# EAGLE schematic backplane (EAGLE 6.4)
AUTHOR: Pat Pannuto; REV: A; TITLE: Signpost Backplane

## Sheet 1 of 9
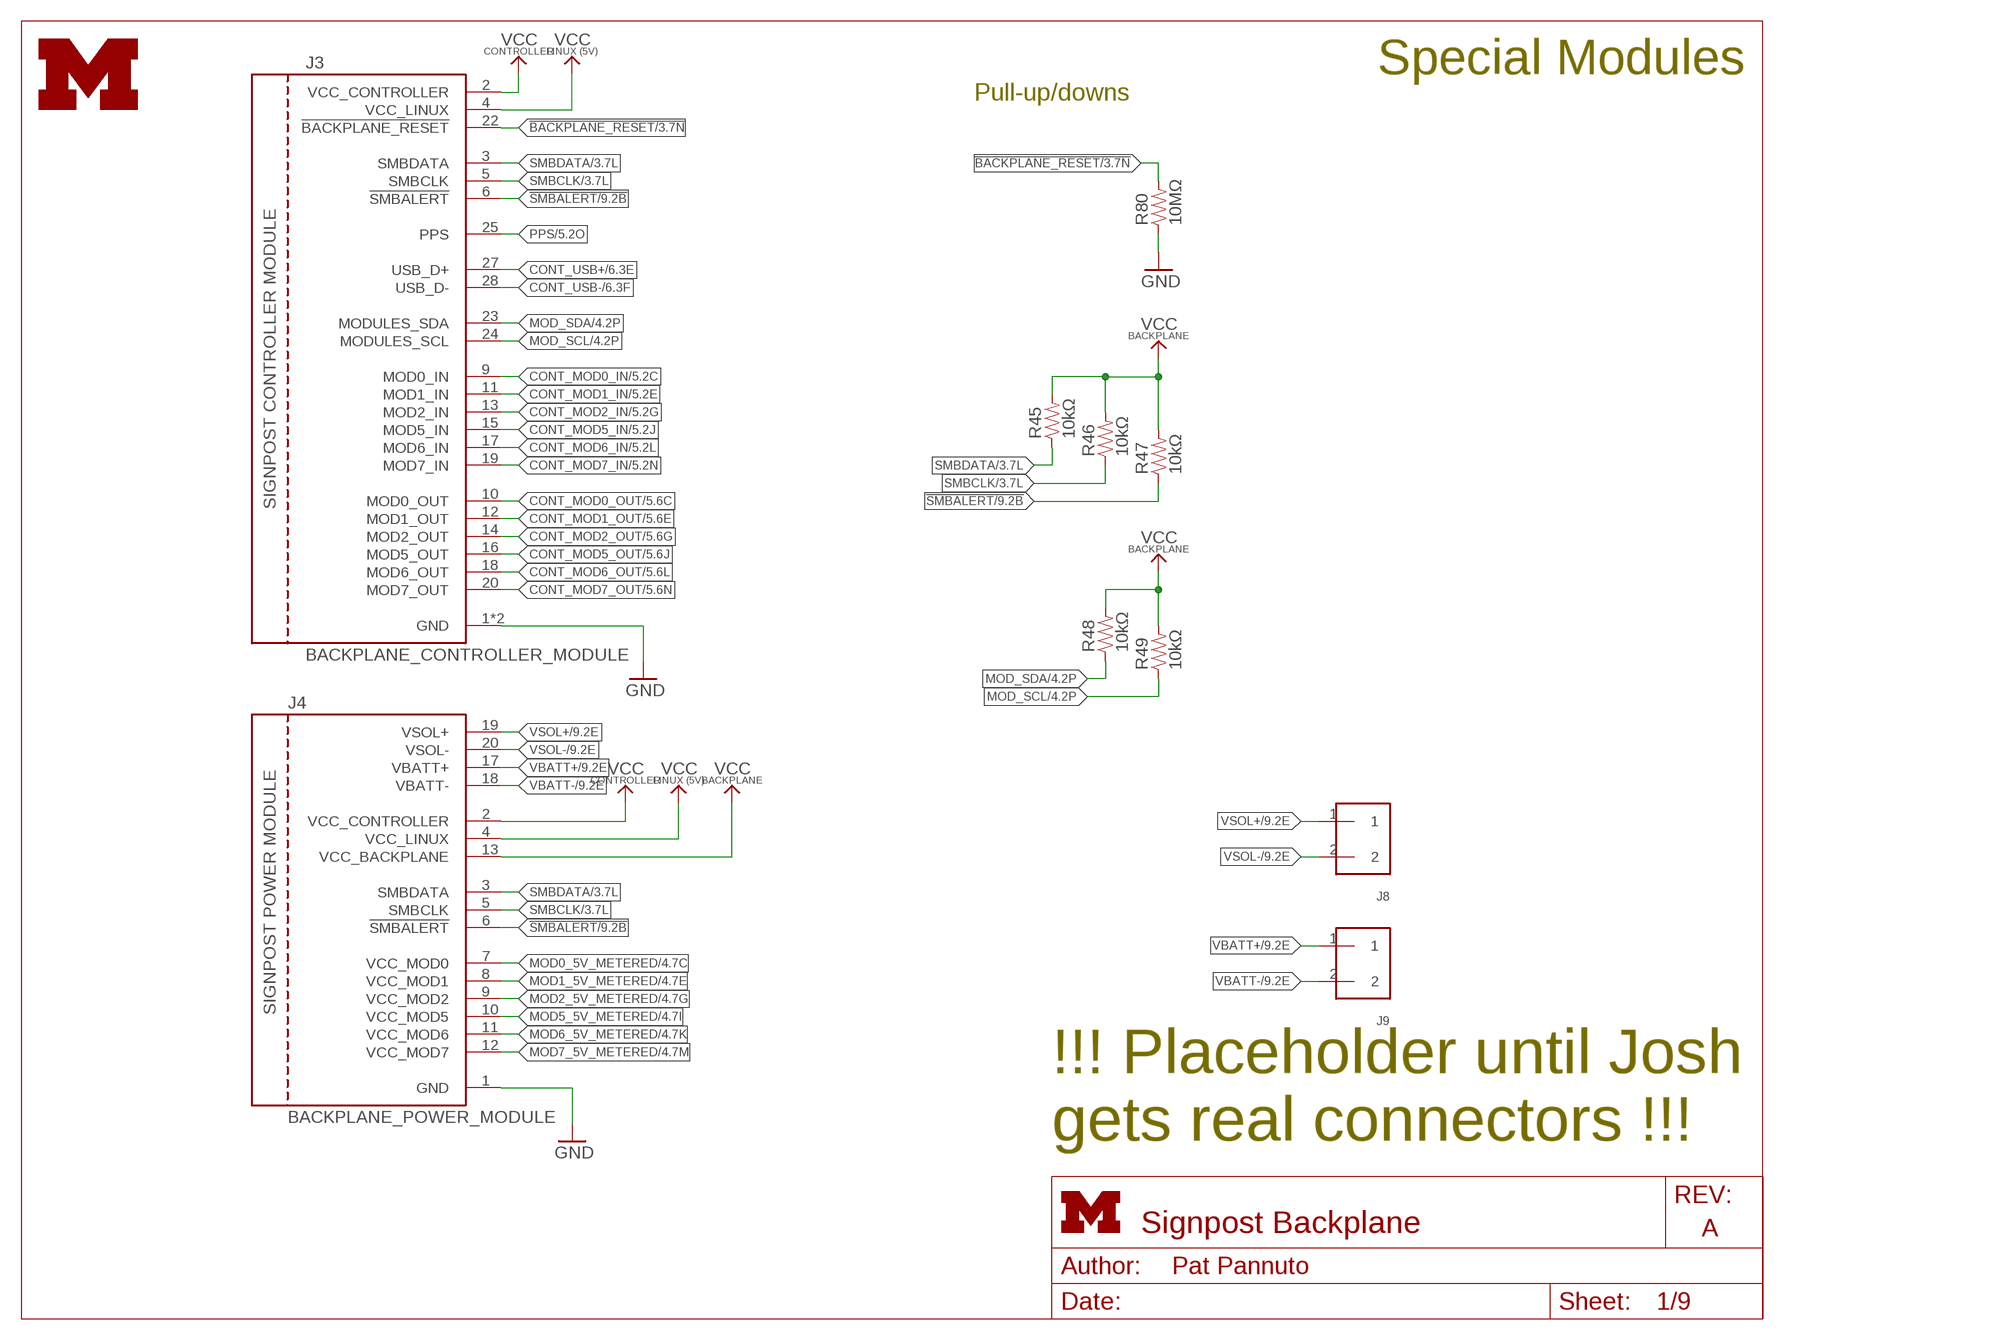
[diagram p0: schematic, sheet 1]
FRAME1 (LETTER_L): HEIGHT: 8.5in; WIDTH: 11in

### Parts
J3  BACKPLANE_CONTROLLER_MODULE  [BACKPLANE_MODULE_20PIN_10PIN]
J4  BACKPLANE_POWER_MODULE  [BACKPLANE_MODULE_20PIN]
J8  SCREW_TERMINAL  [PHEONIX-1935161]
J9  SCREW_TERMINAL  [PHEONIX-1935161]
LOGO1  UMICH_SOLID_GIANT  [UMICH_SOLID_1000MIL]
R45  10kΩ  RESISTOR0603_RES  [0603-RES]
R46  10kΩ  RESISTOR0603_RES  [0603-RES]
R47  10kΩ  RESISTOR0603_RES  [0603-RES]
R48  10kΩ  RESISTOR0603_RES  [0603-RES]
R49  10kΩ  RESISTOR0603_RES  [0603-RES]
R80  10MΩ  RESISTOR0603_RES  [0603-RES]

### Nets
!BACKPLANE_RESET: J3.22(!BACKPLANE_RESET) R80.2 ; also sheet 3,6,9
!SMBALERT: J3.6(!SMBALERT) J4.6(!SMBALERT) R47.1 ; also sheet 9
CONT_MOD0_IN: J3.9(MOD0_IN) ; also sheet 5
CONT_MOD0_OUT: J3.10(MOD0_OUT) ; also sheet 5
CONT_MOD1_IN: J3.11(MOD1_IN) ; also sheet 5
CONT_MOD1_OUT: J3.12(MOD1_OUT) ; also sheet 5
CONT_MOD2_IN: J3.13(MOD2_IN) ; also sheet 5
CONT_MOD2_OUT: J3.14(MOD2_OUT) ; also sheet 5
CONT_MOD5_IN: J3.15(MOD5_IN) ; also sheet 5
CONT_MOD5_OUT: J3.16(MOD5_OUT) ; also sheet 5
CONT_MOD6_IN: J3.17(MOD6_IN) ; also sheet 5
CONT_MOD6_OUT: J3.18(MOD6_OUT) ; also sheet 5
CONT_MOD7_IN: J3.19(MOD7_IN) ; also sheet 5
CONT_MOD7_OUT: J3.20(MOD7_OUT) ; also sheet 5
CONT_USB+: J3.27(USB_D+) ; also sheet 6
CONT_USB-: J3.28(USB_D-) ; also sheet 6
GND: J3.1(GND) J3.21(GND) J4.1(GND) R80.1 ; also sheet 2,3,4,5,6,7,8,9
MOD0_5V_METERED: J4.7(VCC_MOD0) ; also sheet 4,8,9
MOD1_5V_METERED: J4.8(VCC_MOD1) ; also sheet 4,8,9
MOD2_5V_METERED: J4.9(VCC_MOD2) ; also sheet 4,8,9
MOD5_5V_METERED: J4.10(VCC_MOD5) ; also sheet 4,8,9
MOD6_5V_METERED: J4.11(VCC_MOD6) ; also sheet 4,8,9
MOD7_5V_METERED: J4.12(VCC_MOD7) ; also sheet 4,8,9
MOD_SCL: J3.24(MODULES_SCL) R49.1 ; also sheet 4,9
MOD_SDA: J3.23(MODULES_SDA) R48.1 ; also sheet 4,9
PPS: J3.25(PPS) ; also sheet 5,9
SMBCLK: J3.5(SMBCLK) J4.5(SMBCLK) R46.1 ; also sheet 3,9
SMBDATA: J3.3(SMBDATA) J4.3(SMBDATA) R45.1 ; also sheet 3,9
VBATT+: J4.17(VBATT+) J9.1 ; also sheet 9
VBATT-: J4.18(VBATT-) J9.2 ; also sheet 9
VCC_BACKPLANE: J4.13(VCC_BACKPLANE) R45.2 R46.2 R47.2 R48.2 R49.2 ; also sheet 3,4,5,6,7,8,9
VCC_CONTROLLER: J3.2(VCC_CONTROLLER) J4.2(VCC_CONTROLLER) ; also sheet 9
VCC_LINUX: J3.4(VCC_LINUX) J4.4(VCC_LINUX) ; also sheet 9
VSOL+: J4.19(VSOL+) J8.1 ; also sheet 9
VSOL-: J4.20(VSOL-) J8.2 ; also sheet 9

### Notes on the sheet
- Special Modules
- Pull-up/downs
- !!! Placeholder until Josh
  gets real connectors !!!

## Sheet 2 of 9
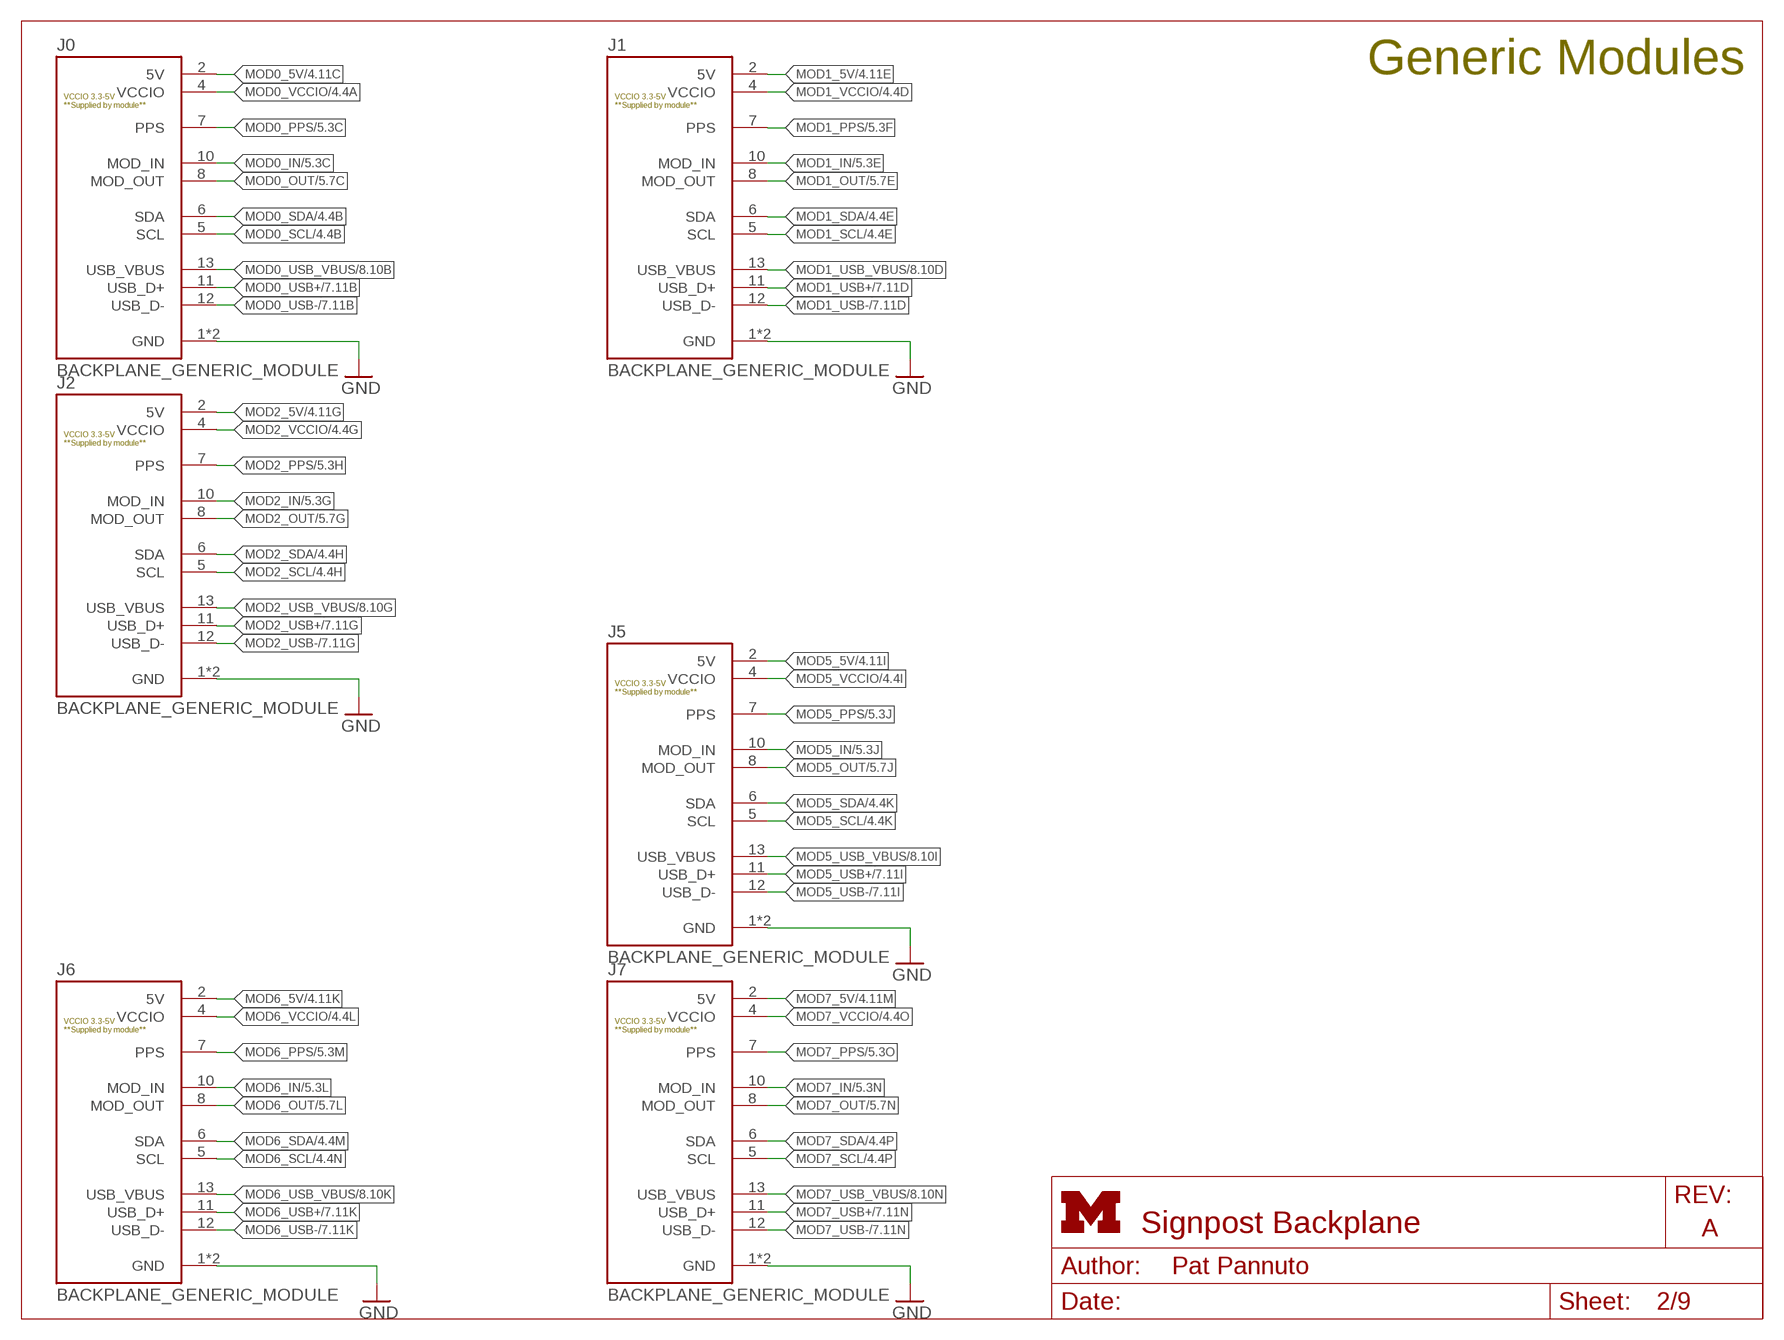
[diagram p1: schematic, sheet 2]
FRAME2 (LETTER_L): HEIGHT: 8.5in; WIDTH: 11in

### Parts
J0  BACKPLANE_GENERIC_MODULE  [BACKPLANE_MODULE_14PIN]
J1  BACKPLANE_GENERIC_MODULE  [BACKPLANE_MODULE_14PIN]
J2  BACKPLANE_GENERIC_MODULE  [BACKPLANE_MODULE_14PIN]
J5  BACKPLANE_GENERIC_MODULE  [BACKPLANE_MODULE_14PIN]
J6  BACKPLANE_GENERIC_MODULE  [BACKPLANE_MODULE_14PIN]
J7  BACKPLANE_GENERIC_MODULE  [BACKPLANE_MODULE_14PIN]

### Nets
GND: J0.1(GND) J0.14(GND) J1.1(GND) J1.14(GND) J2.1(GND) J2.14(GND) J5.1(GND) J5.14(GND) J6.1(GND) J6.14(GND) J7.1(GND) J7.14(GND) ; also sheet 1,3,4,5,6,7,8,9
MOD0_5V: J0.2(5V) ; also sheet 4
MOD0_IN: J0.10(MOD_IN) ; also sheet 5
MOD0_OUT: J0.8(MOD_OUT) ; also sheet 5
MOD0_PPS: J0.7(PPS) ; also sheet 5
MOD0_SCL: J0.5(SCL) ; also sheet 4
MOD0_SDA: J0.6(SDA) ; also sheet 4
MOD0_USB+: J0.11(USB_D+) ; also sheet 7
MOD0_USB-: J0.12(USB_D-) ; also sheet 7
MOD0_USB_VBUS: J0.13(USB_VBUS) ; also sheet 8
MOD0_VCCIO: J0.4(VCCIO) ; also sheet 4,5
MOD1_5V: J1.2(5V) ; also sheet 4
MOD1_IN: J1.10(MOD_IN) ; also sheet 5
MOD1_OUT: J1.8(MOD_OUT) ; also sheet 5
MOD1_PPS: J1.7(PPS) ; also sheet 5
MOD1_SCL: J1.5(SCL) ; also sheet 4
MOD1_SDA: J1.6(SDA) ; also sheet 4
MOD1_USB+: J1.11(USB_D+) ; also sheet 7
MOD1_USB-: J1.12(USB_D-) ; also sheet 7
MOD1_USB_VBUS: J1.13(USB_VBUS) ; also sheet 8
MOD1_VCCIO: J1.4(VCCIO) ; also sheet 4,5
MOD2_5V: J2.2(5V) ; also sheet 4
MOD2_IN: J2.10(MOD_IN) ; also sheet 5
MOD2_OUT: J2.8(MOD_OUT) ; also sheet 5
MOD2_PPS: J2.7(PPS) ; also sheet 5
MOD2_SCL: J2.5(SCL) ; also sheet 4
MOD2_SDA: J2.6(SDA) ; also sheet 4
MOD2_USB+: J2.11(USB_D+) ; also sheet 7
MOD2_USB-: J2.12(USB_D-) ; also sheet 7
MOD2_USB_VBUS: J2.13(USB_VBUS) ; also sheet 8
MOD2_VCCIO: J2.4(VCCIO) ; also sheet 4,5
MOD5_5V: J5.2(5V) ; also sheet 4
MOD5_IN: J5.10(MOD_IN) ; also sheet 5
MOD5_OUT: J5.8(MOD_OUT) ; also sheet 5
MOD5_PPS: J5.7(PPS) ; also sheet 5
MOD5_SCL: J5.5(SCL) ; also sheet 4
MOD5_SDA: J5.6(SDA) ; also sheet 4
MOD5_USB+: J5.11(USB_D+) ; also sheet 7
MOD5_USB-: J5.12(USB_D-) ; also sheet 7
MOD5_USB_VBUS: J5.13(USB_VBUS) ; also sheet 8
MOD5_VCCIO: J5.4(VCCIO) ; also sheet 4,5
MOD6_5V: J6.2(5V) ; also sheet 4
MOD6_IN: J6.10(MOD_IN) ; also sheet 5
MOD6_OUT: J6.8(MOD_OUT) ; also sheet 5
MOD6_PPS: J6.7(PPS) ; also sheet 5
MOD6_SCL: J6.5(SCL) ; also sheet 4
MOD6_SDA: J6.6(SDA) ; also sheet 4
MOD6_USB+: J6.11(USB_D+) ; also sheet 7
MOD6_USB-: J6.12(USB_D-) ; also sheet 7
MOD6_USB_VBUS: J6.13(USB_VBUS) ; also sheet 8
MOD6_VCCIO: J6.4(VCCIO) ; also sheet 4,5
MOD7_5V: J7.2(5V) ; also sheet 4
MOD7_IN: J7.10(MOD_IN) ; also sheet 5
MOD7_OUT: J7.8(MOD_OUT) ; also sheet 5
MOD7_PPS: J7.7(PPS) ; also sheet 5
MOD7_SCL: J7.5(SCL) ; also sheet 4
MOD7_SDA: J7.6(SDA) ; also sheet 4
MOD7_USB+: J7.11(USB_D+) ; also sheet 7
MOD7_USB-: J7.12(USB_D-) ; also sheet 7
MOD7_USB_VBUS: J7.13(USB_VBUS) ; also sheet 8
MOD7_VCCIO: J7.4(VCCIO) ; also sheet 4,5

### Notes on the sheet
- Generic Modules

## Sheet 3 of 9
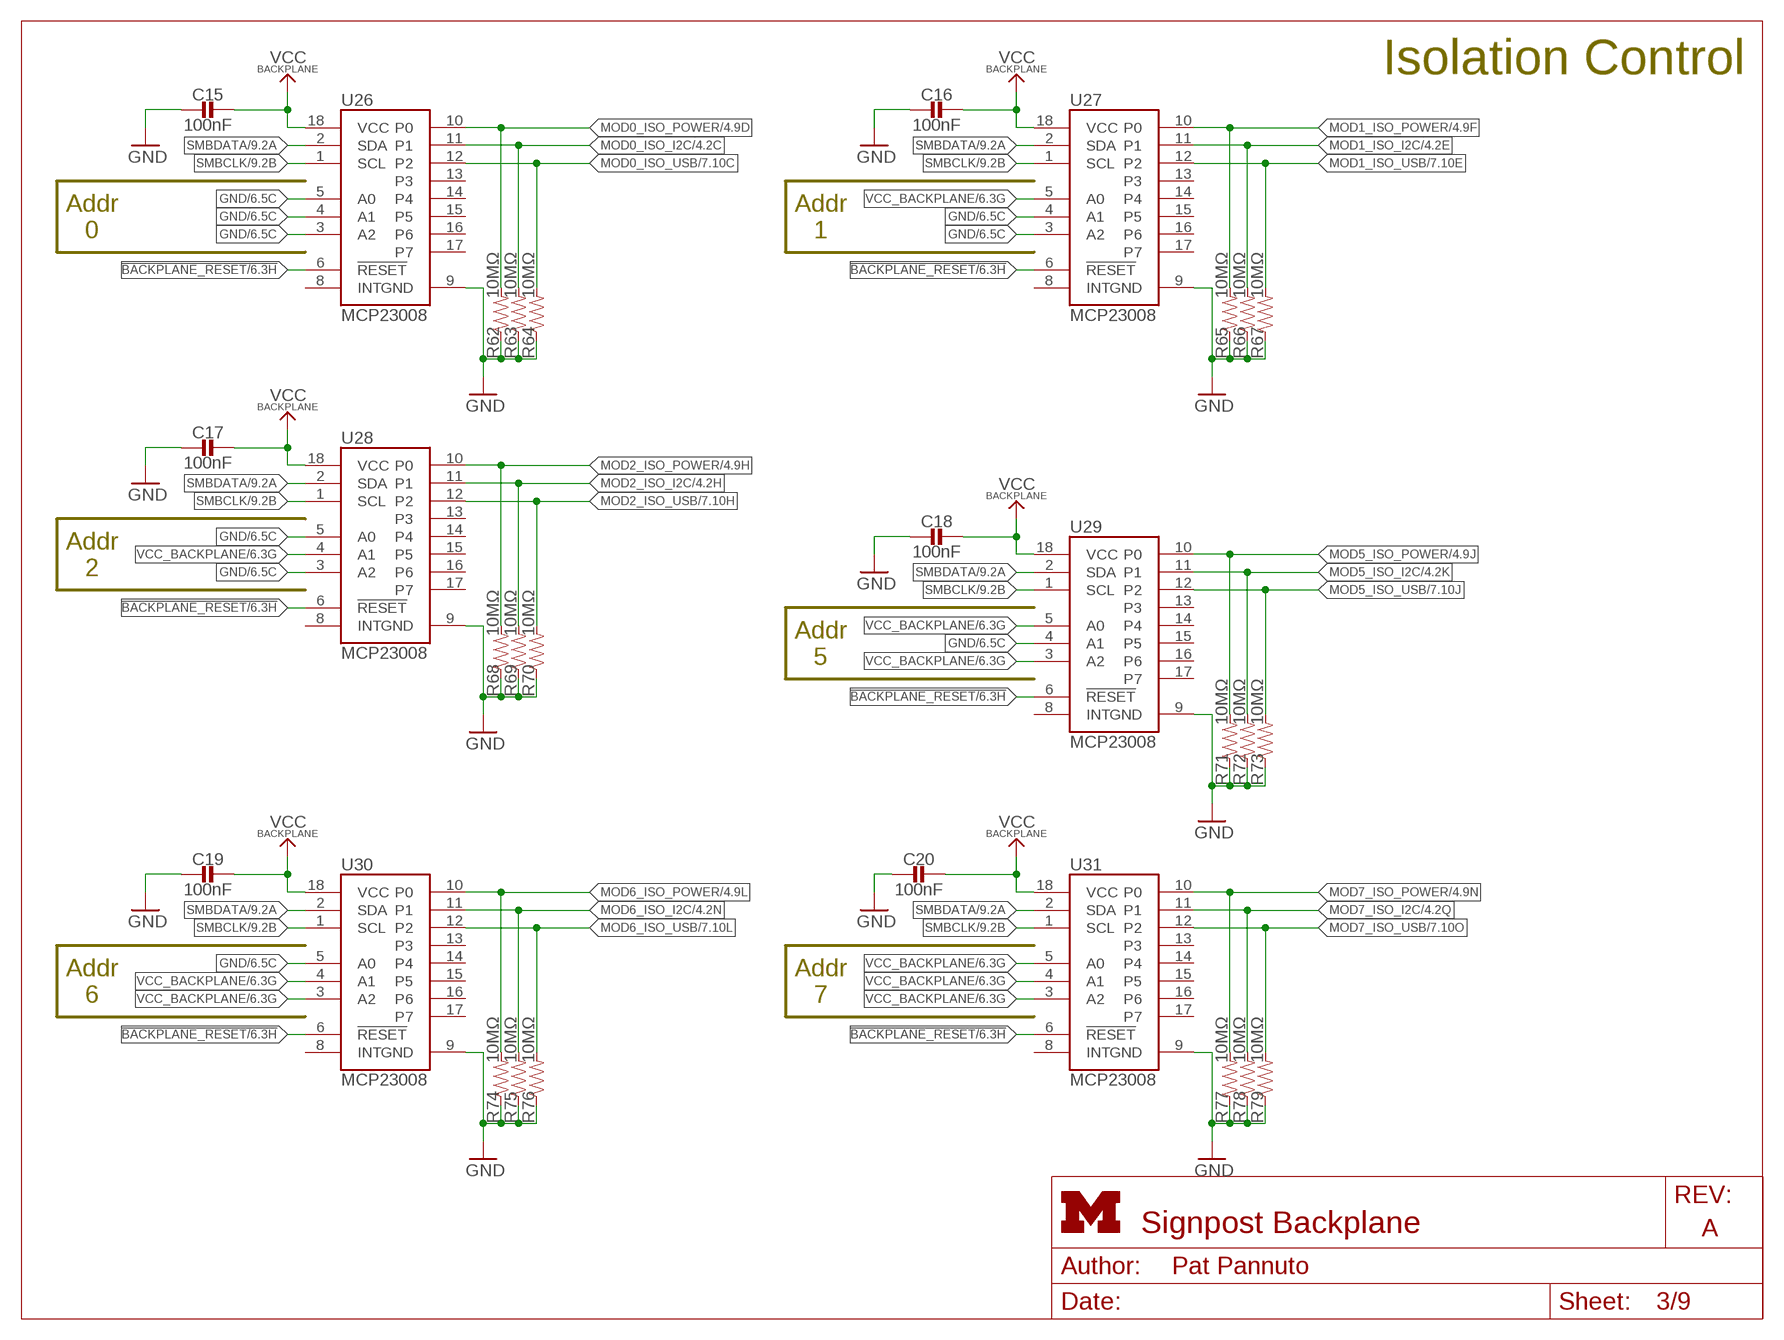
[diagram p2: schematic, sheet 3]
FRAME7 (LETTER_L_UMICH): HEIGHT: 8.5in; WIDTH: 11in

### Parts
C15  100nF  CAPACITOR0603_CAP  [0603_CAP]
C16  100nF  CAPACITOR0603_CAP  [0603_CAP]
C17  100nF  CAPACITOR0603_CAP  [0603_CAP]
C18  100nF  CAPACITOR0603_CAP  [0603_CAP]
C19  100nF  CAPACITOR0603_CAP  [0603_CAP]
C20  100nF  CAPACITOR0603_CAP  [0603_CAP]
R62  10MΩ  RESISTOR0603_RES  [0603-RES]
R63  10MΩ  RESISTOR0603_RES  [0603-RES]
R64  10MΩ  RESISTOR0603_RES  [0603-RES]
R65  10MΩ  RESISTOR0603_RES  [0603-RES]
R66  10MΩ  RESISTOR0603_RES  [0603-RES]
R67  10MΩ  RESISTOR0603_RES  [0603-RES]
R68  10MΩ  RESISTOR0603_RES  [0603-RES]
R69  10MΩ  RESISTOR0603_RES  [0603-RES]
R70  10MΩ  RESISTOR0603_RES  [0603-RES]
R71  10MΩ  RESISTOR0603_RES  [0603-RES]
R72  10MΩ  RESISTOR0603_RES  [0603-RES]
R73  10MΩ  RESISTOR0603_RES  [0603-RES]
R74  10MΩ  RESISTOR0603_RES  [0603-RES]
R75  10MΩ  RESISTOR0603_RES  [0603-RES]
R76  10MΩ  RESISTOR0603_RES  [0603-RES]
R77  10MΩ  RESISTOR0603_RES  [0603-RES]
R78  10MΩ  RESISTOR0603_RES  [0603-RES]
R79  10MΩ  RESISTOR0603_RES  [0603-RES]
U26  MCP23008  [SOIC-18]
U27  MCP23008  [SOIC-18]
U28  MCP23008  [SOIC-18]
U29  MCP23008  [SOIC-18]
U30  MCP23008  [SOIC-18]
U31  MCP23008  [SOIC-18]

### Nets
!BACKPLANE_RESET: U26.6(!RESET) U27.6(!RESET) U28.6(!RESET) U29.6(!RESET) U30.6(!RESET) U31.6(!RESET) ; also sheet 1,6,9
GND: C15.2 C16.2 C17.2 C18.2 C19.2 C20.2 R62.1 R63.1 R64.1 R65.1 R66.1 R67.1 R68.1 R69.1 R70.1 R71.1 R72.1 R73.1 R74.1 R75.1 R76.1 R77.1 R78.1 R79.1 U26.3(A2) U26.4(A1) U26.5(A0) U26.9(GND) U27.3(A2) U27.4(A1) U27.9(GND) U28.3(A2) U28.5(A0) U28.9(GND) U29.4(A1) U29.9(GND) U30.5(A0) U30.9(GND) U31.9(GND) ; also sheet 1,2,4,5,6,7,8,9
MOD0_ISO_I2C: R63.2 U26.11(P1) ; also sheet 4,9
MOD0_ISO_POWER: R62.2 U26.10(P0) ; also sheet 4,9
MOD0_ISO_USB: R64.2 U26.12(P2) ; also sheet 7,8,9
MOD1_ISO_I2C: R66.2 U27.11(P1) ; also sheet 4,9
MOD1_ISO_POWER: R65.2 U27.10(P0) ; also sheet 4,9
MOD1_ISO_USB: R67.2 U27.12(P2) ; also sheet 7,8,9
MOD2_ISO_I2C: R69.2 U28.11(P1) ; also sheet 4,9
MOD2_ISO_POWER: R68.2 U28.10(P0) ; also sheet 4,9
MOD2_ISO_USB: R70.2 U28.12(P2) ; also sheet 7,8,9
MOD5_ISO_I2C: R72.2 U29.11(P1) ; also sheet 4,9
MOD5_ISO_POWER: R71.2 U29.10(P0) ; also sheet 4,9
MOD5_ISO_USB: R73.2 U29.12(P2) ; also sheet 7,8,9
MOD6_ISO_I2C: R75.2 U30.11(P1) ; also sheet 4,9
MOD6_ISO_POWER: R74.2 U30.10(P0) ; also sheet 4,9
MOD6_ISO_USB: R76.2 U30.12(P2) ; also sheet 7,8,9
MOD7_ISO_I2C: R78.2 U31.11(P1) ; also sheet 4,9
MOD7_ISO_POWER: R77.2 U31.10(P0) ; also sheet 4,9
MOD7_ISO_USB: R79.2 U31.12(P2) ; also sheet 7,8,9
SMBCLK: U26.1(SCL) U27.1(SCL) U28.1(SCL) U29.1(SCL) U30.1(SCL) U31.1(SCL) ; also sheet 1,9
SMBDATA: U26.2(SDA) U27.2(SDA) U28.2(SDA) U29.2(SDA) U30.2(SDA) U31.2(SDA) ; also sheet 1,9
VCC_BACKPLANE: C15.1 C16.1 C17.1 C18.1 C19.1 C20.1 U26.18(VCC) U27.5(A0) U27.18(VCC) U28.4(A1) U28.18(VCC) U29.3(A2) U29.5(A0) U29.18(VCC) U30.3(A2) U30.4(A1) U30.18(VCC) U31.3(A2) U31.4(A1) U31.5(A0) U31.18(VCC) ; also sheet 1,4,5,6,7,8,9
Unconnected: U26.8(INT) U26.13(P3) U26.14(P4) U26.15(P5) U26.16(P6) U26.17(P7) U27.8(INT) U27.13(P3) U27.14(P4) U27.15(P5) U27.16(P6) U27.17(P7) U28.8(INT) U28.13(P3) U28.14(P4) U28.15(P5) U28.16(P6) U28.17(P7) U29.8(INT) U29.13(P3) U29.14(P4) U29.15(P5) U29.16(P6) U29.17(P7) U30.8(INT) U30.13(P3) U30.14(P4) U30.15(P5) U30.16(P6) U30.17(P7) U31.8(INT) U31.13(P3) U31.14(P4) U31.15(P5) U31.16(P6) U31.17(P7)

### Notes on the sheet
- Isolation Control
- Addr
  0
- Addr
  1
- Addr
  2
- Addr
  5
- Addr
  6
- Addr
  7

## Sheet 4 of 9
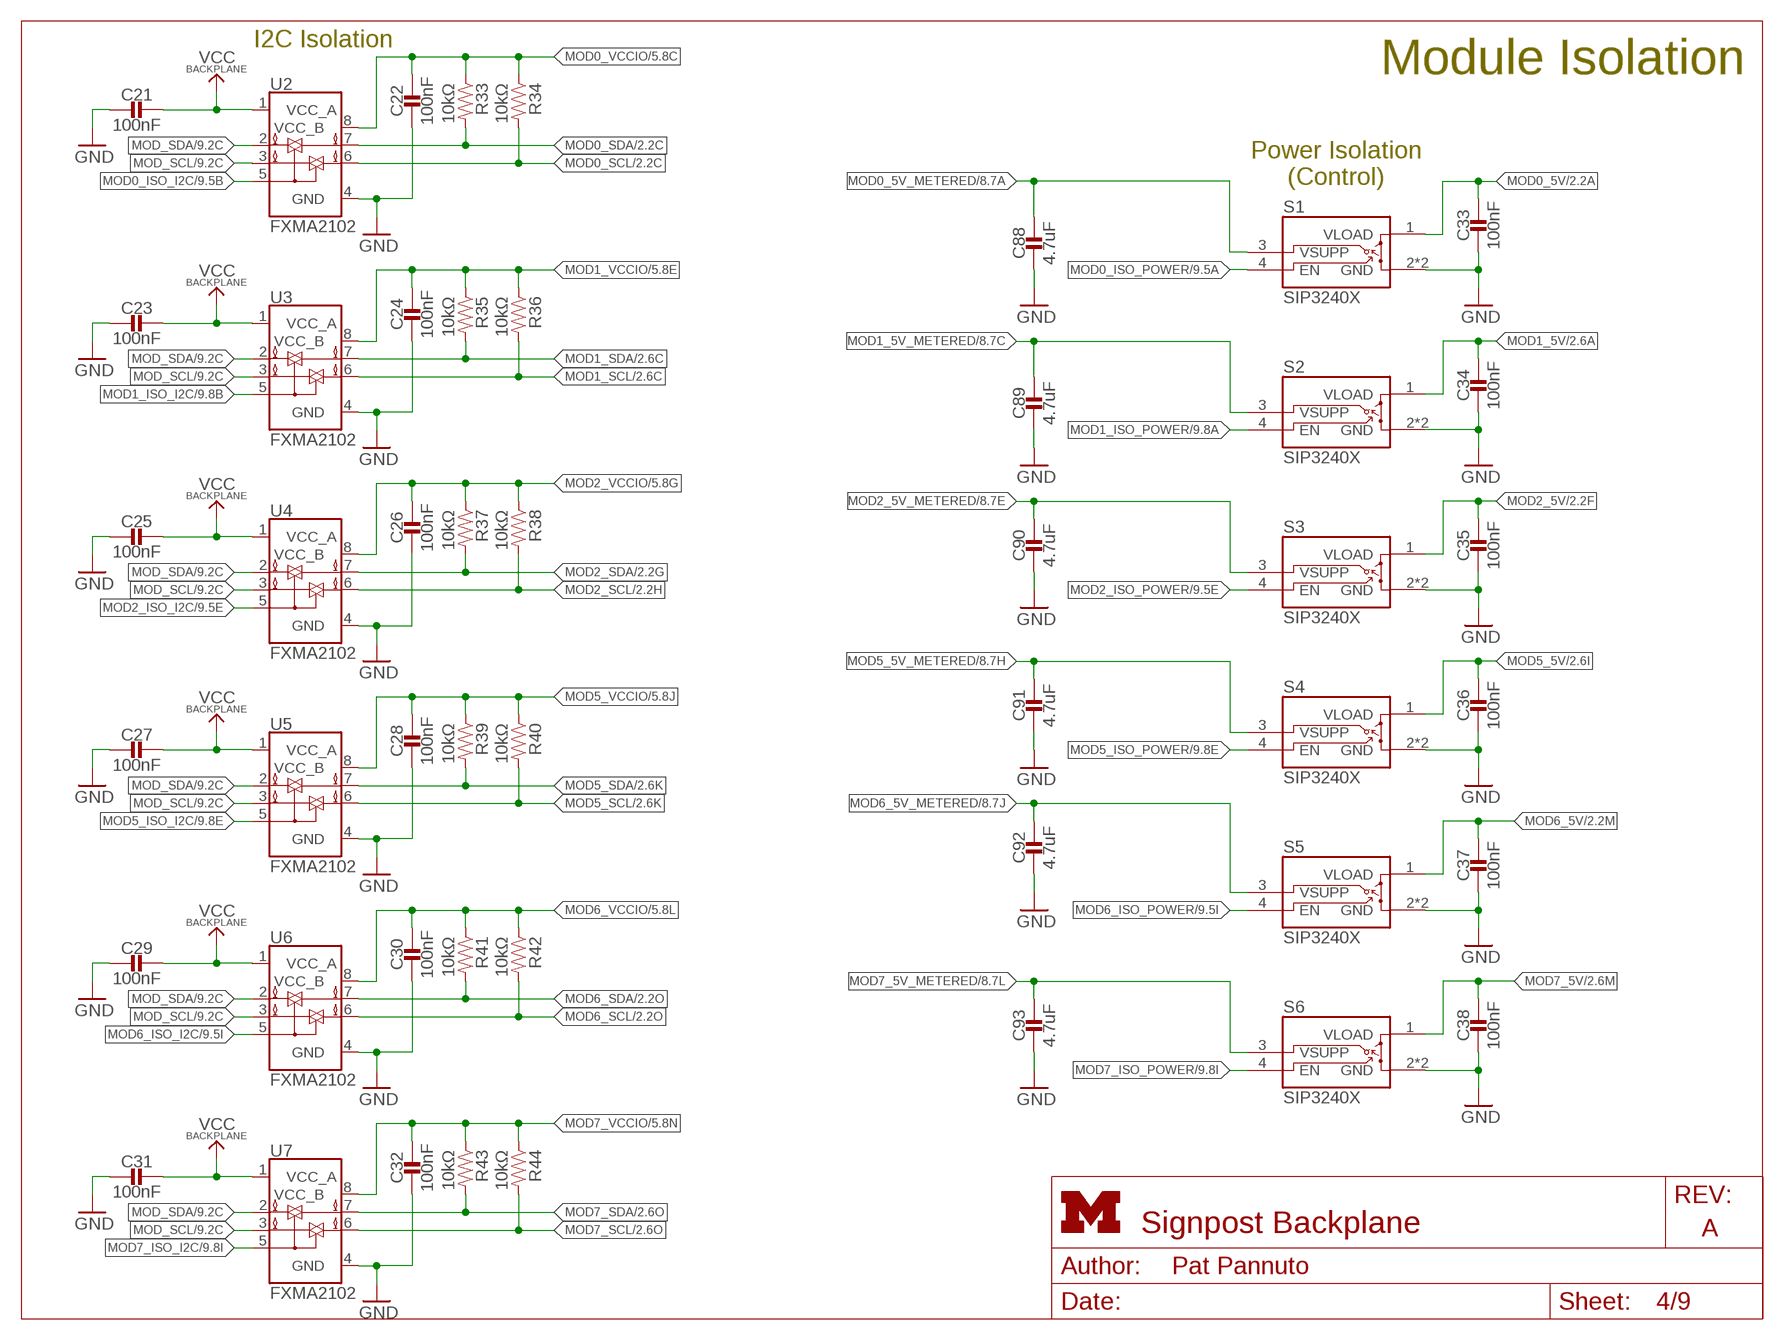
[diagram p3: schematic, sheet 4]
FRAME4 (LETTER_L): HEIGHT: 8.5in; WIDTH: 11in

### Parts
C21  100nF  CAPACITOR0603_CAP  [0603_CAP]
C22  100nF  CAPACITOR0603_CAP  [0603_CAP]
C23  100nF  CAPACITOR0603_CAP  [0603_CAP]
C24  100nF  CAPACITOR0603_CAP  [0603_CAP]
C25  100nF  CAPACITOR0603_CAP  [0603_CAP]
C26  100nF  CAPACITOR0603_CAP  [0603_CAP]
C27  100nF  CAPACITOR0603_CAP  [0603_CAP]
C28  100nF  CAPACITOR0603_CAP  [0603_CAP]
C29  100nF  CAPACITOR0603_CAP  [0603_CAP]
C30  100nF  CAPACITOR0603_CAP  [0603_CAP]
C31  100nF  CAPACITOR0603_CAP  [0603_CAP]
C32  100nF  CAPACITOR0603_CAP  [0603_CAP]
C33  100nF  CAPACITOR0603_CAP  [0603_CAP]
C34  100nF  CAPACITOR0603_CAP  [0603_CAP]
C35  100nF  CAPACITOR0603_CAP  [0603_CAP]
C36  100nF  CAPACITOR0603_CAP  [0603_CAP]
C37  100nF  CAPACITOR0603_CAP  [0603_CAP]
C38  100nF  CAPACITOR0603_CAP  [0603_CAP]
C88  4.7uF  CAPACITOR0603_CAP  [0603_CAP]
C89  4.7uF  CAPACITOR0603_CAP  [0603_CAP]
C90  4.7uF  CAPACITOR0603_CAP  [0603_CAP]
C91  4.7uF  CAPACITOR0603_CAP  [0603_CAP]
C92  4.7uF  CAPACITOR0603_CAP  [0603_CAP]
C93  4.7uF  CAPACITOR0603_CAP  [0603_CAP]
R33  10kΩ  RESISTOR0603_RES  [0603-RES]
R34  10kΩ  RESISTOR0603_RES  [0603-RES]
R35  10kΩ  RESISTOR0603_RES  [0603-RES]
R36  10kΩ  RESISTOR0603_RES  [0603-RES]
R37  10kΩ  RESISTOR0603_RES  [0603-RES]
R38  10kΩ  RESISTOR0603_RES  [0603-RES]
R39  10kΩ  RESISTOR0603_RES  [0603-RES]
R40  10kΩ  RESISTOR0603_RES  [0603-RES]
R41  10kΩ  RESISTOR0603_RES  [0603-RES]
R42  10kΩ  RESISTOR0603_RES  [0603-RES]
R43  10kΩ  RESISTOR0603_RES  [0603-RES]
R44  10kΩ  RESISTOR0603_RES  [0603-RES]
S1  SIP3240X  [TDFN4]
S2  SIP3240X  [TDFN4]
S3  SIP3240X  [TDFN4]
S4  SIP3240X  [TDFN4]
S5  SIP3240X  [TDFN4]
S6  SIP3240X  [TDFN4]
U2  FXMA2102  [UMLP-8]
U3  FXMA2102  [UMLP-8]
U4  FXMA2102  [UMLP-8]
U5  FXMA2102  [UMLP-8]
U6  FXMA2102  [UMLP-8]
U7  FXMA2102  [UMLP-8]

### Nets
GND: C21.2 C22.2 C23.2 C24.2 C25.2 C26.2 C27.2 C28.2 C29.2 C30.2 C31.2 C32.2 C33.2 C34.2 C35.2 C36.2 C37.2 C38.2 C88.2 C89.2 C90.2 C91.2 C92.2 C93.2 S1.2(GND) S1.PAD(GND) S2.2(GND) S2.PAD(GND) S3.2(GND) S3.PAD(GND) S4.2(GND) S4.PAD(GND) S5.2(GND) S5.PAD(GND) S6.2(GND) S6.PAD(GND) U2.4(GND) U3.4(GND) U4.4(GND) U5.4(GND) U6.4(GND) U7.4(GND) ; also sheet 1,2,3,5,6,7,8,9
MOD0_5V: C33.1 S1.1(VLOAD) ; also sheet 2
MOD0_5V_METERED: C88.1 S1.3(VSUPP) ; also sheet 1,8,9
MOD0_ISO_I2C: U2.5(OE) ; also sheet 3,9
MOD0_ISO_POWER: S1.4(EN) ; also sheet 3,9
MOD0_SCL: R34.2 U2.6(B1) ; also sheet 2
MOD0_SDA: R33.2 U2.7(B0) ; also sheet 2
MOD0_VCCIO: C22.1 R33.1 R34.1 U2.8(VCC_B) ; also sheet 2,5
MOD1_5V: C34.1 S2.1(VLOAD) ; also sheet 2
MOD1_5V_METERED: C89.1 S2.3(VSUPP) ; also sheet 1,8,9
MOD1_ISO_I2C: U3.5(OE) ; also sheet 3,9
MOD1_ISO_POWER: S2.4(EN) ; also sheet 3,9
MOD1_SCL: R36.2 U3.6(B1) ; also sheet 2
MOD1_SDA: R35.2 U3.7(B0) ; also sheet 2
MOD1_VCCIO: C24.1 R35.1 R36.1 U3.8(VCC_B) ; also sheet 2,5
MOD2_5V: C35.1 S3.1(VLOAD) ; also sheet 2
MOD2_5V_METERED: C90.1 S3.3(VSUPP) ; also sheet 1,8,9
MOD2_ISO_I2C: U4.5(OE) ; also sheet 3,9
MOD2_ISO_POWER: S3.4(EN) ; also sheet 3,9
MOD2_SCL: R38.2 U4.6(B1) ; also sheet 2
MOD2_SDA: R37.2 U4.7(B0) ; also sheet 2
MOD2_VCCIO: C26.1 R37.1 R38.1 U4.8(VCC_B) ; also sheet 2,5
MOD5_5V: C36.1 S4.1(VLOAD) ; also sheet 2
MOD5_5V_METERED: C91.1 S4.3(VSUPP) ; also sheet 1,8,9
MOD5_ISO_I2C: U5.5(OE) ; also sheet 3,9
MOD5_ISO_POWER: S4.4(EN) ; also sheet 3,9
MOD5_SCL: R40.2 U5.6(B1) ; also sheet 2
MOD5_SDA: R39.2 U5.7(B0) ; also sheet 2
MOD5_VCCIO: C28.1 R39.1 R40.1 U5.8(VCC_B) ; also sheet 2,5
MOD6_5V: C37.1 S5.1(VLOAD) ; also sheet 2
MOD6_5V_METERED: C92.1 S5.3(VSUPP) ; also sheet 1,8,9
MOD6_ISO_I2C: U6.5(OE) ; also sheet 3,9
MOD6_ISO_POWER: S5.4(EN) ; also sheet 3,9
MOD6_SCL: R42.2 U6.6(B1) ; also sheet 2
MOD6_SDA: R41.2 U6.7(B0) ; also sheet 2
MOD6_VCCIO: C30.1 R41.1 R42.1 U6.8(VCC_B) ; also sheet 2,5
MOD7_5V: C38.1 S6.1(VLOAD) ; also sheet 2
MOD7_5V_METERED: C93.1 S6.3(VSUPP) ; also sheet 1,8,9
MOD7_ISO_I2C: U7.5(OE) ; also sheet 3,9
MOD7_ISO_POWER: S6.4(EN) ; also sheet 3,9
MOD7_SCL: R44.2 U7.6(B1) ; also sheet 2
MOD7_SDA: R43.2 U7.7(B0) ; also sheet 2
MOD7_VCCIO: C32.1 R43.1 R44.1 U7.8(VCC_B) ; also sheet 2,5
MOD_SCL: U2.3(A1) U3.3(A1) U4.3(A1) U5.3(A1) U6.3(A1) U7.3(A1) ; also sheet 1,9
MOD_SDA: U2.2(A0) U3.2(A0) U4.2(A0) U5.2(A0) U6.2(A0) U7.2(A0) ; also sheet 1,9
VCC_BACKPLANE: C21.1 C23.1 C25.1 C27.1 C29.1 C31.1 U2.1(VCC_A) U3.1(VCC_A) U4.1(VCC_A) U5.1(VCC_A) U6.1(VCC_A) U7.1(VCC_A) ; also sheet 1,3,5,6,7,8,9

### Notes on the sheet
- I2C Isolation | Module Isolation
- Power Isolation
  (Control)

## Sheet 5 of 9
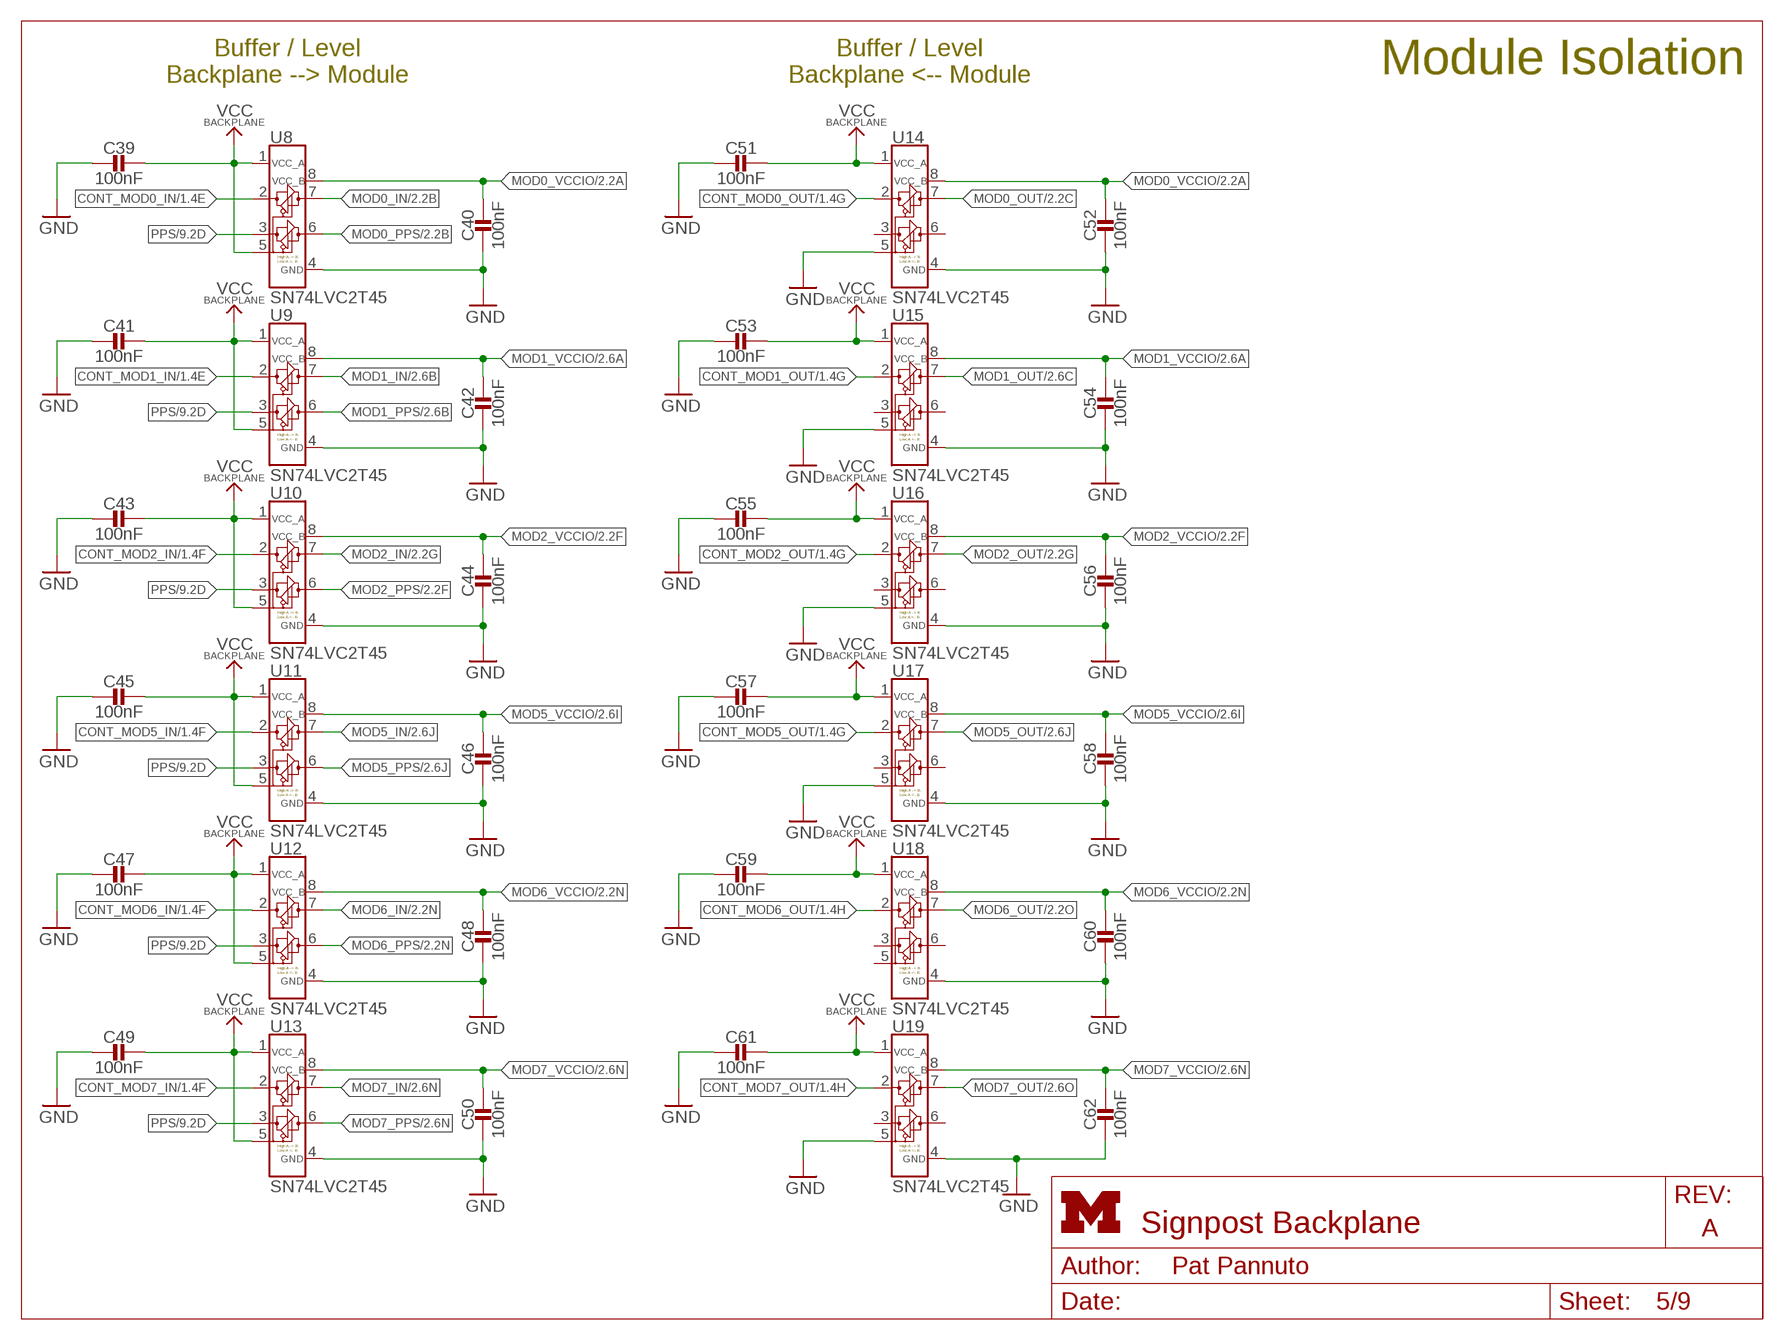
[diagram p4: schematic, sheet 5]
FRAME5 (LETTER_L_UMICH): HEIGHT: 8.5in; WIDTH: 11in

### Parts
C39  100nF  CAPACITOR0603_CAP  [0603_CAP]
C40  100nF  CAPACITOR0603_CAP  [0603_CAP]
C41  100nF  CAPACITOR0603_CAP  [0603_CAP]
C42  100nF  CAPACITOR0603_CAP  [0603_CAP]
C43  100nF  CAPACITOR0603_CAP  [0603_CAP]
C44  100nF  CAPACITOR0603_CAP  [0603_CAP]
C45  100nF  CAPACITOR0603_CAP  [0603_CAP]
C46  100nF  CAPACITOR0603_CAP  [0603_CAP]
C47  100nF  CAPACITOR0603_CAP  [0603_CAP]
C48  100nF  CAPACITOR0603_CAP  [0603_CAP]
C49  100nF  CAPACITOR0603_CAP  [0603_CAP]
C50  100nF  CAPACITOR0603_CAP  [0603_CAP]
C51  100nF  CAPACITOR0603_CAP  [0603_CAP]
C52  100nF  CAPACITOR0603_CAP  [0603_CAP]
C53  100nF  CAPACITOR0603_CAP  [0603_CAP]
C54  100nF  CAPACITOR0603_CAP  [0603_CAP]
C55  100nF  CAPACITOR0603_CAP  [0603_CAP]
C56  100nF  CAPACITOR0603_CAP  [0603_CAP]
C57  100nF  CAPACITOR0603_CAP  [0603_CAP]
C58  100nF  CAPACITOR0603_CAP  [0603_CAP]
C59  100nF  CAPACITOR0603_CAP  [0603_CAP]
C60  100nF  CAPACITOR0603_CAP  [0603_CAP]
C61  100nF  CAPACITOR0603_CAP  [0603_CAP]
C62  100nF  CAPACITOR0603_CAP  [0603_CAP]
U8  SN74LVC2T45  [VFSOP-8]
U9  SN74LVC2T45  [VFSOP-8]
U10  SN74LVC2T45  [VFSOP-8]
U11  SN74LVC2T45  [VFSOP-8]
U12  SN74LVC2T45  [VFSOP-8]
U13  SN74LVC2T45  [VFSOP-8]
U14  SN74LVC2T45  [VFSOP-8]
U15  SN74LVC2T45  [VFSOP-8]
U16  SN74LVC2T45  [VFSOP-8]
U17  SN74LVC2T45  [VFSOP-8]
U18  SN74LVC2T45  [VFSOP-8]
U19  SN74LVC2T45  [VFSOP-8]

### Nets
CONT_MOD0_IN: U8.2(A1) ; also sheet 1
CONT_MOD0_OUT: U14.2(A1) ; also sheet 1
CONT_MOD1_IN: U9.2(A1) ; also sheet 1
CONT_MOD1_OUT: U15.2(A1) ; also sheet 1
CONT_MOD2_IN: U10.2(A1) ; also sheet 1
CONT_MOD2_OUT: U16.2(A1) ; also sheet 1
CONT_MOD5_IN: U11.2(A1) ; also sheet 1
CONT_MOD5_OUT: U17.2(A1) ; also sheet 1
CONT_MOD6_IN: U12.2(A1) ; also sheet 1
CONT_MOD6_OUT: U18.2(A1) ; also sheet 1
CONT_MOD7_IN: U13.2(A1) ; also sheet 1
CONT_MOD7_OUT: U19.2(A1) ; also sheet 1
GND: C39.2 C40.2 C41.2 C42.2 C43.2 C44.2 C45.2 C46.2 C47.2 C48.2 C49.2 C50.2 C51.2 C52.2 C53.2 C54.2 C55.2 C56.2 C57.2 C58.2 C59.2 C60.2 C61.2 C62.2 U8.4(GND) U9.4(GND) U10.4(GND) U11.4(GND) U12.4(GND) U13.4(GND) U14.4(GND) U14.5(DIR) U15.4(GND) U15.5(DIR) U16.4(GND) U16.5(DIR) U17.4(GND) U17.5(DIR) U18.4(GND) U19.4(GND) U19.5(DIR) ; also sheet 1,2,3,4,6,7,8,9
MOD0_IN: U8.7(B1) ; also sheet 2
MOD0_OUT: U14.7(B1) ; also sheet 2
MOD0_PPS: U8.6(B2) ; also sheet 2
MOD0_VCCIO: C40.1 C52.1 U8.8(VCC_B) U14.8(VCC_B) ; also sheet 2,4
MOD1_IN: U9.7(B1) ; also sheet 2
MOD1_OUT: U15.7(B1) ; also sheet 2
MOD1_PPS: U9.6(B2) ; also sheet 2
MOD1_VCCIO: C42.1 C54.1 U9.8(VCC_B) U15.8(VCC_B) ; also sheet 2,4
MOD2_IN: U10.7(B1) ; also sheet 2
MOD2_OUT: U16.7(B1) ; also sheet 2
MOD2_PPS: U10.6(B2) ; also sheet 2
MOD2_VCCIO: C44.1 C56.1 U10.8(VCC_B) U16.8(VCC_B) ; also sheet 2,4
MOD5_IN: U11.7(B1) ; also sheet 2
MOD5_OUT: U17.7(B1) ; also sheet 2
MOD5_PPS: U11.6(B2) ; also sheet 2
MOD5_VCCIO: C46.1 C58.1 U11.8(VCC_B) U17.8(VCC_B) ; also sheet 2,4
MOD6_IN: U12.7(B1) ; also sheet 2
MOD6_OUT: U18.7(B1) ; also sheet 2
MOD6_PPS: U12.6(B2) ; also sheet 2
MOD6_VCCIO: C48.1 C60.1 U12.8(VCC_B) U18.8(VCC_B) ; also sheet 2,4
MOD7_IN: U13.7(B1) ; also sheet 2
MOD7_OUT: U19.7(B1) ; also sheet 2
MOD7_PPS: U13.6(B2) ; also sheet 2
MOD7_VCCIO: C50.1 C62.1 U13.8(VCC_B) U19.8(VCC_B) ; also sheet 2,4
PPS: U8.3(A2) U9.3(A2) U10.3(A2) U11.3(A2) U12.3(A2) U13.3(A2) ; also sheet 1,9
VCC_BACKPLANE: C39.1 C41.1 C43.1 C45.1 C47.1 C49.1 C51.1 C53.1 C55.1 C57.1 C59.1 C61.1 U8.1(VCC_A) U8.5(DIR) U9.1(VCC_A) U9.5(DIR) U10.1(VCC_A) U10.5(DIR) U11.1(VCC_A) U11.5(DIR) U12.1(VCC_A) U12.5(DIR) U13.1(VCC_A) U13.5(DIR) U14.1(VCC_A) U15.1(VCC_A) U16.1(VCC_A) U17.1(VCC_A) U18.1(VCC_A) U19.1(VCC_A) ; also sheet 1,3,4,6,7,8,9
Unconnected: U14.3(A2) U14.6(B2) U15.3(A2) U15.6(B2) U16.3(A2) U16.6(B2) U17.3(A2) U17.6(B2) U18.3(A2) U18.5(DIR) U18.6(B2) U19.3(A2) U19.6(B2)

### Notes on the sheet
- Buffer / Level
  Backplane --> Module
- Buffer / Level
  Backplane <-- Module
- Module Isolation

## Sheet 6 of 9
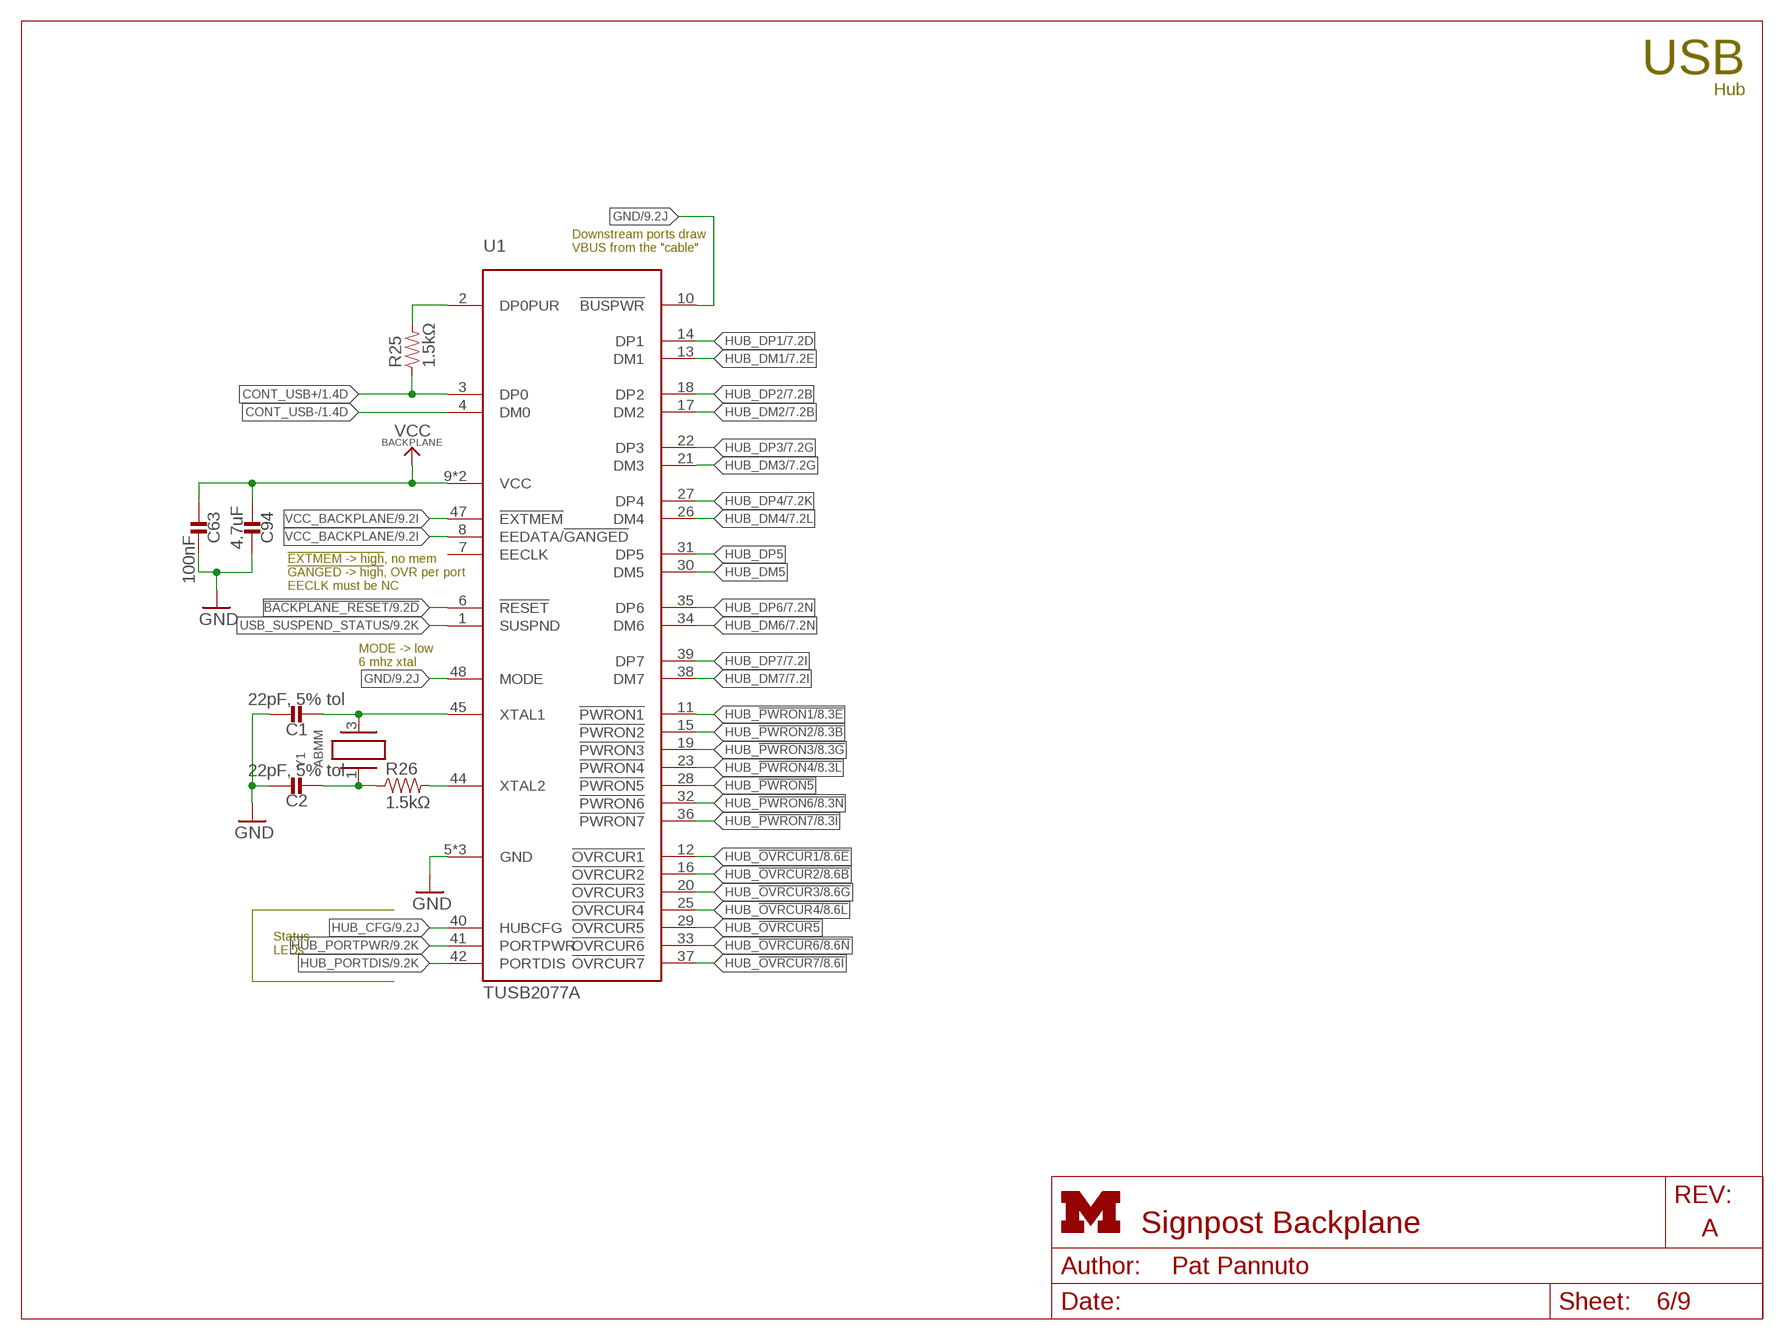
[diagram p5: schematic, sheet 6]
FRAME8 (LETTER_L_UMICH): HEIGHT: 8.5in; WIDTH: 11in

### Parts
C1  22pF, 5% tol  CAPACITOR0603_CAP  [0603_CAP]
C2  22pF, 5% tol  CAPACITOR0603_CAP  [0603_CAP]
C63  100nF  CAPACITOR0603_CAP  [0603_CAP]
C94  4.7uF  CAPACITOR0603_CAP  [0603_CAP]
R25  1.5kΩ  RESISTOR0603_RES  [0603-RES]
R26  1.5kΩ  RESISTOR0603_RES  [0603-RES]
U1  TUSB2077A  [LQFP-48]
Y1  ABMM  [ABMM]

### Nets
!BACKPLANE_RESET: U1.6(!RESET) ; also sheet 1,3,9
CONT_USB+: R25.1 U1.3(DP0) ; also sheet 1
CONT_USB-: U1.4(DM0) ; also sheet 1
GND: C1.1 C2.1 C63.1 C94.1 U1.5(GND) U1.10(!BUSPWR) U1.24(GND) U1.43(GND) U1.48(MODE) ; also sheet 1,2,3,4,5,7,8,9
HUB_!OVRCUR1: U1.12(!OVRCUR1) ; also sheet 8,9
HUB_!OVRCUR2: U1.16(!OVRCUR2) ; also sheet 8,9
HUB_!OVRCUR3: U1.20(!OVRCUR3) ; also sheet 8,9
HUB_!OVRCUR4: U1.25(!OVRCUR4) ; also sheet 8,9
HUB_!OVRCUR5: U1.29(!OVRCUR5)
HUB_!OVRCUR6: U1.33(!OVRCUR6) ; also sheet 8,9
HUB_!OVRCUR7: U1.37(!OVRCUR7) ; also sheet 8,9
HUB_!PWRON1: U1.11(!PWRON1) ; also sheet 8,9
HUB_!PWRON2: U1.15(!PWRON2) ; also sheet 8,9
HUB_!PWRON3: U1.19(!PWRON3) ; also sheet 8,9
HUB_!PWRON4: U1.23(!PWRON4) ; also sheet 8,9
HUB_!PWRON5: U1.28(!PWRON5)
HUB_!PWRON6: U1.32(!PWRON6) ; also sheet 8,9
HUB_!PWRON7: U1.36(!PWRON7) ; also sheet 8,9
HUB_CFG: U1.40(HUBCFG) ; also sheet 9
HUB_DM1: U1.13(DM1) ; also sheet 7
HUB_DM2: U1.17(DM2) ; also sheet 7
HUB_DM3: U1.21(DM3) ; also sheet 7
HUB_DM4: U1.26(DM4) ; also sheet 7
HUB_DM5: U1.30(DM5)
HUB_DM6: U1.34(DM6) ; also sheet 7
HUB_DM7: U1.38(DM7) ; also sheet 7
HUB_DP1: U1.14(DP1) ; also sheet 7
HUB_DP2: U1.18(DP2) ; also sheet 7
HUB_DP3: U1.22(DP3) ; also sheet 7
HUB_DP4: U1.27(DP4) ; also sheet 7
HUB_DP5: U1.31(DP5)
HUB_DP6: U1.35(DP6) ; also sheet 7
HUB_DP7: U1.39(DP7) ; also sheet 7
HUB_PORTDIS: U1.42(PORTDIS) ; also sheet 9
HUB_PORTPWR: U1.41(PORTPWR) ; also sheet 9
N$12: R25.2 U1.2(DP0PUR)
N$14: C2.2 R26.1 Y1.1
N$73: C1.2 U1.45(XTAL1) Y1.3
N$74: R26.2 U1.44(XTAL2)
USB_SUSPEND_STATUS: U1.1(SUSPND) ; also sheet 9
VCC_BACKPLANE: C63.2 C94.2 U1.8(EEDATA/!GANGED) U1.9(VCC) U1.46(VCC) U1.47(!EXTMEM) ; also sheet 1,3,4,5,7,8,9
Unconnected: U1.7(EECLK)

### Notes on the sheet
- USB
- Hub
- Downstream ports draw
  VBUS from the "cable"
- !EXTMEM -> high, no mem
  !GANGED -> high, OVR per port
  EECLK must be NC
- MODE -> low
  6 mhz xtal
- Status
  LEDs

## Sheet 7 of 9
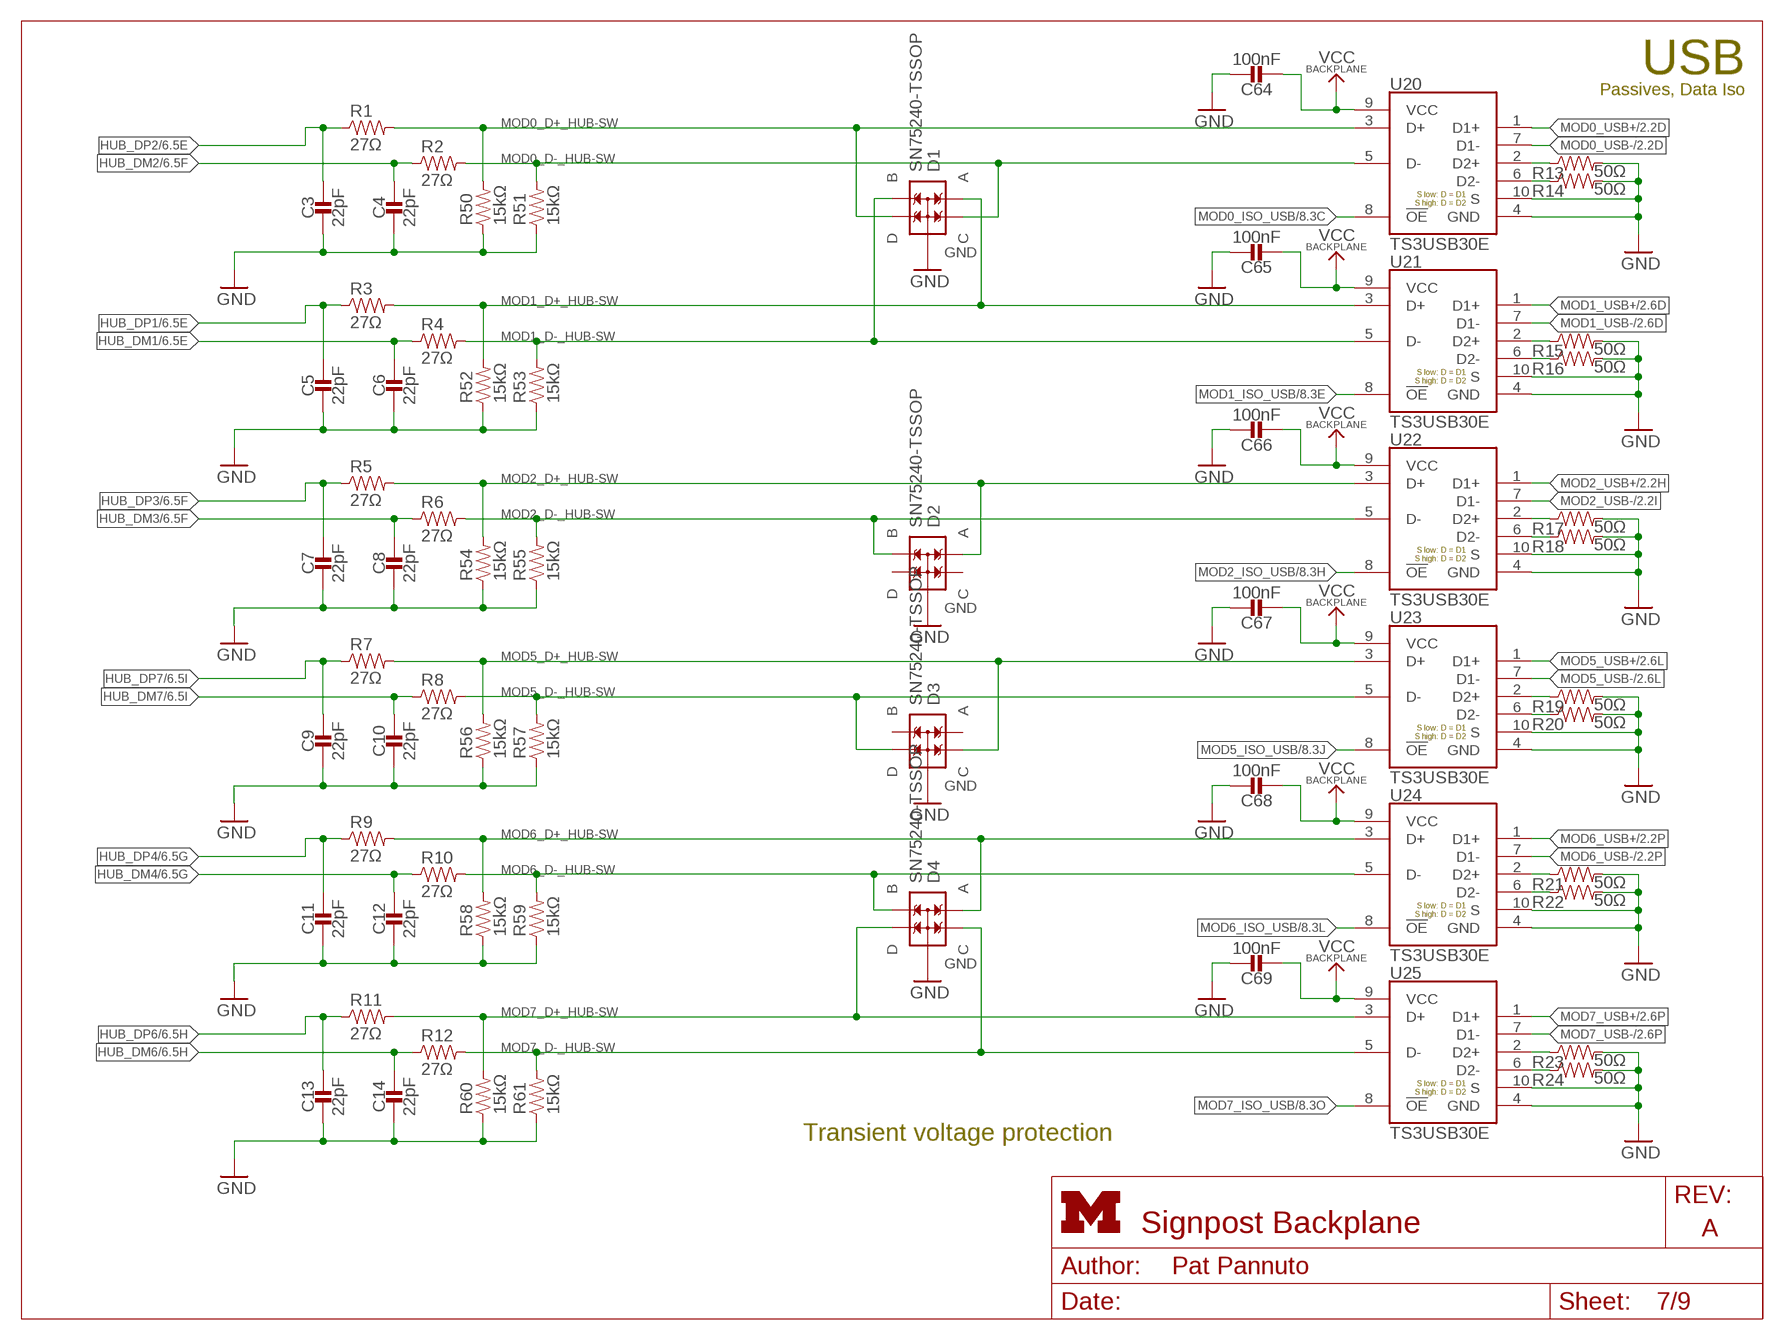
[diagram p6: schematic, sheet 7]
FRAME3 (LETTER_L): HEIGHT: 8.5in; WIDTH: 11in

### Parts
C3  22pF  CAPACITOR0402_CAP  [0402_CAP]
C4  22pF  CAPACITOR0402_CAP  [0402_CAP]
C5  22pF  CAPACITOR0402_CAP  [0402_CAP]
C6  22pF  CAPACITOR0402_CAP  [0402_CAP]
C7  22pF  CAPACITOR0402_CAP  [0402_CAP]
C8  22pF  CAPACITOR0402_CAP  [0402_CAP]
C9  22pF  CAPACITOR0402_CAP  [0402_CAP]
C10  22pF  CAPACITOR0402_CAP  [0402_CAP]
C11  22pF  CAPACITOR0402_CAP  [0402_CAP]
C12  22pF  CAPACITOR0402_CAP  [0402_CAP]
C13  22pF  CAPACITOR0402_CAP  [0402_CAP]
C14  22pF  CAPACITOR0402_CAP  [0402_CAP]
C64  100nF  CAPACITOR0603_CAP  [0603_CAP]
C65  100nF  CAPACITOR0603_CAP  [0603_CAP]
C66  100nF  CAPACITOR0603_CAP  [0603_CAP]
C67  100nF  CAPACITOR0603_CAP  [0603_CAP]
C68  100nF  CAPACITOR0603_CAP  [0603_CAP]
C69  100nF  CAPACITOR0603_CAP  [0603_CAP]
D1  SN75240-TSSOP  [TSSOP-8]
D2  SN75240-TSSOP  [TSSOP-8]
D3  SN75240-TSSOP  [TSSOP-8]
D4  SN75240-TSSOP  [TSSOP-8]
R1  27Ω  RESISTOR0402_RES-HIGH_SPEED  [0402_RES-HIGH_SPEED]
R2  27Ω  RESISTOR0402_RES-HIGH_SPEED  [0402_RES-HIGH_SPEED]
R3  27Ω  RESISTOR0402_RES-HIGH_SPEED  [0402_RES-HIGH_SPEED]
R4  27Ω  RESISTOR0402_RES-HIGH_SPEED  [0402_RES-HIGH_SPEED]
R5  27Ω  RESISTOR0402_RES-HIGH_SPEED  [0402_RES-HIGH_SPEED]
R6  27Ω  RESISTOR0402_RES-HIGH_SPEED  [0402_RES-HIGH_SPEED]
R7  27Ω  RESISTOR0402_RES-HIGH_SPEED  [0402_RES-HIGH_SPEED]
R8  27Ω  RESISTOR0402_RES-HIGH_SPEED  [0402_RES-HIGH_SPEED]
R9  27Ω  RESISTOR0402_RES-HIGH_SPEED  [0402_RES-HIGH_SPEED]
R10  27Ω  RESISTOR0402_RES-HIGH_SPEED  [0402_RES-HIGH_SPEED]
R11  27Ω  RESISTOR0402_RES-HIGH_SPEED  [0402_RES-HIGH_SPEED]
R12  27Ω  RESISTOR0402_RES-HIGH_SPEED  [0402_RES-HIGH_SPEED]
R13  50Ω  RESISTOR0603_RES  [0603-RES]
R14  50Ω  RESISTOR0603_RES  [0603-RES]
R15  50Ω  RESISTOR0603_RES  [0603-RES]
R16  50Ω  RESISTOR0603_RES  [0603-RES]
R17  50Ω  RESISTOR0603_RES  [0603-RES]
R18  50Ω  RESISTOR0603_RES  [0603-RES]
R19  50Ω  RESISTOR0603_RES  [0603-RES]
R20  50Ω  RESISTOR0603_RES  [0603-RES]
R21  50Ω  RESISTOR0603_RES  [0603-RES]
R22  50Ω  RESISTOR0603_RES  [0603-RES]
R23  50Ω  RESISTOR0603_RES  [0603-RES]
R24  50Ω  RESISTOR0603_RES  [0603-RES]
R50  15kΩ  RESISTOR0603_RES  [0603-RES]
R51  15kΩ  RESISTOR0603_RES  [0603-RES]
R52  15kΩ  RESISTOR0603_RES  [0603-RES]
R53  15kΩ  RESISTOR0603_RES  [0603-RES]
R54  15kΩ  RESISTOR0603_RES  [0603-RES]
R55  15kΩ  RESISTOR0603_RES  [0603-RES]
R56  15kΩ  RESISTOR0603_RES  [0603-RES]
R57  15kΩ  RESISTOR0603_RES  [0603-RES]
R58  15kΩ  RESISTOR0603_RES  [0603-RES]
R59  15kΩ  RESISTOR0603_RES  [0603-RES]
R60  15kΩ  RESISTOR0603_RES  [0603-RES]
R61  15kΩ  RESISTOR0603_RES  [0603-RES]
U20  TS3USB30E  [UQFN-10]
U21  TS3USB30E  [UQFN-10]
U22  TS3USB30E  [UQFN-10]
U23  TS3USB30E  [UQFN-10]
U24  TS3USB30E  [UQFN-10]
U25  TS3USB30E  [UQFN-10]

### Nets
GND: C3.2 C4.2 C5.2 C6.2 C7.2 C8.2 C9.2 C10.2 C11.2 C12.2 C13.2 C14.2 C64.1 C65.1 C66.1 C67.1 C68.1 C69.1 D1.1(GND) D1.3(GND) D1.5(GND) D1.7(GND) D2.1(GND) D2.3(GND) D2.5(GND) D2.7(GND) D3.1(GND) D3.3(GND) D3.5(GND) D3.7(GND) D4.1(GND) D4.3(GND) D4.5(GND) D4.7(GND) R13.2 R14.2 R15.2 R16.2 R17.2 R18.2 R19.2 R20.2 R21.2 R22.2 R23.2 R24.2 R50.1 R51.1 R52.1 R53.1 R54.1 R55.1 R56.1 R57.1 R58.1 R59.1 R60.1 R61.1 U20.4(GND) U20.10(S) U21.4(GND) U21.10(S) U22.4(GND) U22.10(S) U23.4(GND) U23.10(S) U24.4(GND) U24.10(S) U25.4(GND) U25.10(S) ; also sheet 1,2,3,4,5,6,8,9
HUB_DM1: C6.1 R4.1 ; also sheet 6
HUB_DM2: C4.1 R2.1 ; also sheet 6
HUB_DM3: C8.1 R6.1 ; also sheet 6
HUB_DM4: C12.1 R10.1 ; also sheet 6
HUB_DM6: C14.1 R12.1 ; also sheet 6
HUB_DM7: C10.1 R8.1 ; also sheet 6
HUB_DP1: C5.1 R3.1 ; also sheet 6
HUB_DP2: C3.1 R1.1 ; also sheet 6
HUB_DP3: C7.1 R5.1 ; also sheet 6
HUB_DP4: C11.1 R9.1 ; also sheet 6
HUB_DP6: C13.1 R11.1 ; also sheet 6
HUB_DP7: C9.1 R7.1 ; also sheet 6
MOD0_D+_HUB-SW: D1.4(D) R1.2 R50.2 U20.3(D+)
MOD0_D-_HUB-SW: D1.2(C) R2.2 R51.2 U20.5(D-)
MOD0_ISO_USB: U20.8(!OE) ; also sheet 3,8,9
MOD0_USB+: U20.1(D1+) ; also sheet 2
MOD0_USB-: U20.7(D1-) ; also sheet 2
MOD1_D+_HUB-SW: D1.8(A) R3.2 R52.2 U21.3(D+)
MOD1_D-_HUB-SW: D1.6(B) R4.2 R53.2 U21.5(D-)
MOD1_ISO_USB: U21.8(!OE) ; also sheet 3,8,9
MOD1_USB+: U21.1(D1+) ; also sheet 2
MOD1_USB-: U21.7(D1-) ; also sheet 2
MOD2_D+_HUB-SW: D2.8(A) R5.2 R54.2 U22.3(D+)
MOD2_D-_HUB-SW: D2.6(B) R6.2 R55.2 U22.5(D-)
MOD2_ISO_USB: U22.8(!OE) ; also sheet 3,8,9
MOD2_USB+: U22.1(D1+) ; also sheet 2
MOD2_USB-: U22.7(D1-) ; also sheet 2
MOD5_D+_HUB-SW: D3.2(C) R7.2 R56.2 U23.3(D+)
MOD5_D-_HUB-SW: D3.4(D) R8.2 R57.2 U23.5(D-)
MOD5_ISO_USB: U23.8(!OE) ; also sheet 3,8,9
MOD5_USB+: U23.1(D1+) ; also sheet 2
MOD5_USB-: U23.7(D1-) ; also sheet 2
MOD6_D+_HUB-SW: D4.8(A) R9.2 R58.2 U24.3(D+)
MOD6_D-_HUB-SW: D4.6(B) R10.2 R59.2 U24.5(D-)
MOD6_ISO_USB: U24.8(!OE) ; also sheet 3,8,9
MOD6_USB+: U24.1(D1+) ; also sheet 2
MOD6_USB-: U24.7(D1-) ; also sheet 2
MOD7_D+_HUB-SW: D4.4(D) R11.2 R60.2 U25.3(D+)
MOD7_D-_HUB-SW: D4.2(C) R12.2 R61.2 U25.5(D-)
MOD7_ISO_USB: U25.8(!OE) ; also sheet 3,8,9
MOD7_USB+: U25.1(D1+) ; also sheet 2
MOD7_USB-: U25.7(D1-) ; also sheet 2
N$17: R13.1 U20.2(D2+)
N$18: R24.1 U25.6(D2-)
N$19: R23.1 U25.2(D2+)
N$20: R22.1 U24.6(D2-)
N$21: R21.1 U24.2(D2+)
N$22: R20.1 U23.6(D2-)
N$23: R19.1 U23.2(D2+)
N$24: R17.1 U22.2(D2+)
N$25: R18.1 U22.6(D2-)
N$26: R16.1 U21.6(D2-)
N$27: R15.1 U21.2(D2+)
N$31: R14.1 U20.6(D2-)
VCC_BACKPLANE: C64.2 C65.2 C66.2 C67.2 C68.2 C69.2 U20.9(VCC) U21.9(VCC) U22.9(VCC) U23.9(VCC) U24.9(VCC) U25.9(VCC) ; also sheet 1,3,4,5,6,8,9
Unconnected: D2.2(C) D2.4(D) D3.6(B) D3.8(A)

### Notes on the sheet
- USB
- Passives, Data Iso
- Transient voltage protection

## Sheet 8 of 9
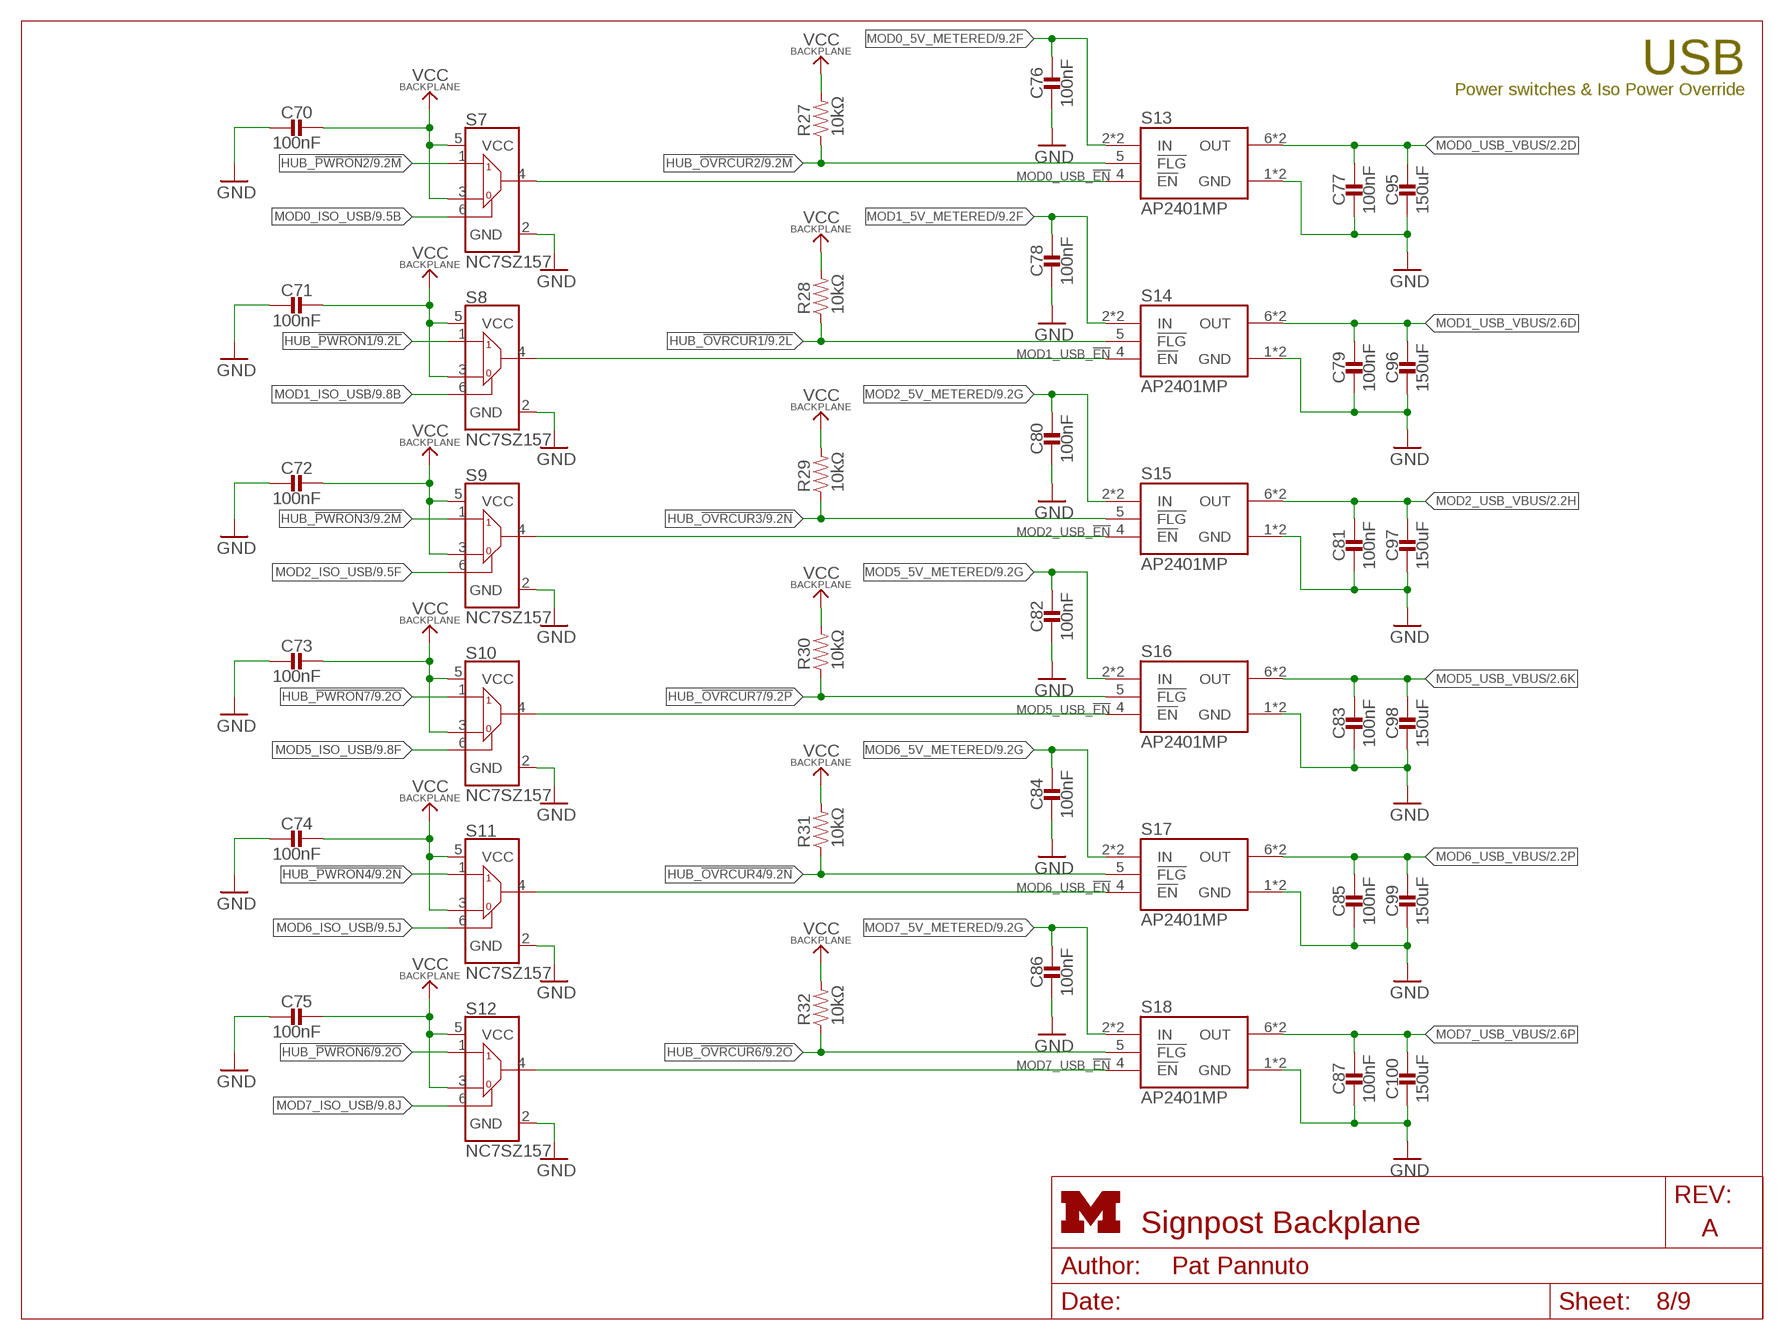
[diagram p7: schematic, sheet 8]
FRAME6 (LETTER_L_UMICH): HEIGHT: 8.5in; WIDTH: 11in

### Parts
C70  100nF  CAPACITOR0603_CAP  [0603_CAP]
C71  100nF  CAPACITOR0603_CAP  [0603_CAP]
C72  100nF  CAPACITOR0603_CAP  [0603_CAP]
C73  100nF  CAPACITOR0603_CAP  [0603_CAP]
C74  100nF  CAPACITOR0603_CAP  [0603_CAP]
C75  100nF  CAPACITOR0603_CAP  [0603_CAP]
C76  100nF  CAPACITOR0603_CAP  [0603_CAP]
C77  100nF  CAPACITOR0603_CAP  [0603_CAP]
C78  100nF  CAPACITOR0603_CAP  [0603_CAP]
C79  100nF  CAPACITOR0603_CAP  [0603_CAP]
C80  100nF  CAPACITOR0603_CAP  [0603_CAP]
C81  100nF  CAPACITOR0603_CAP  [0603_CAP]
C82  100nF  CAPACITOR0603_CAP  [0603_CAP]
C83  100nF  CAPACITOR0603_CAP  [0603_CAP]
C84  100nF  CAPACITOR0603_CAP  [0603_CAP]
C85  100nF  CAPACITOR0603_CAP  [0603_CAP]
C86  100nF  CAPACITOR0603_CAP  [0603_CAP]
C87  100nF  CAPACITOR0603_CAP  [0603_CAP]
C95  150uF  CAPACITOR1210_CAP  [1210_CAP]
C96  150uF  CAPACITOR1210_CAP  [1210_CAP]
C97  150uF  CAPACITOR1210_CAP  [1210_CAP]
C98  150uF  CAPACITOR1210_CAP  [1210_CAP]
C99  150uF  CAPACITOR1210_CAP  [1210_CAP]
C100  150uF  CAPACITOR1210_CAP  [1210_CAP]
R27  10kΩ  RESISTOR0603_RES  [0603-RES]
R28  10kΩ  RESISTOR0603_RES  [0603-RES]
R29  10kΩ  RESISTOR0603_RES  [0603-RES]
R30  10kΩ  RESISTOR0603_RES  [0603-RES]
R31  10kΩ  RESISTOR0603_RES  [0603-RES]
R32  10kΩ  RESISTOR0603_RES  [0603-RES]
S7  NC7SZ157  [SC70-6]
S8  NC7SZ157  [SC70-6]
S9  NC7SZ157  [SC70-6]
S10  NC7SZ157  [SC70-6]
S11  NC7SZ157  [SC70-6]
S12  NC7SZ157  [SC70-6]
S13  AP2401MP  [MSOP-8EP]
S14  AP2401MP  [MSOP-8EP]
S15  AP2401MP  [MSOP-8EP]
S16  AP2401MP  [MSOP-8EP]
S17  AP2401MP  [MSOP-8EP]
S18  AP2401MP  [MSOP-8EP]

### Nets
GND: C70.2 C71.2 C72.2 C73.2 C74.2 C75.2 C76.2 C77.2 C78.2 C79.2 C80.2 C81.2 C82.2 C83.2 C84.2 C85.2 C86.2 C87.2 C95.2 C96.2 C97.2 C98.2 C99.2 C100.2 S7.2(GND) S8.2(GND) S9.2(GND) S10.2(GND) S11.2(GND) S12.2(GND) S13.1(GND) S13.PAD(GND) S14.1(GND) S14.PAD(GND) S15.1(GND) S15.PAD(GND) S16.1(GND) S16.PAD(GND) S17.1(GND) S17.PAD(GND) S18.1(GND) S18.PAD(GND) ; also sheet 1,2,3,4,5,6,7,9
HUB_!OVRCUR1: R28.1 S14.5(!FLG) ; also sheet 6,9
HUB_!OVRCUR2: R27.1 S13.5(!FLG) ; also sheet 6,9
HUB_!OVRCUR3: R29.1 S15.5(!FLG) ; also sheet 6,9
HUB_!OVRCUR4: R31.1 S17.5(!FLG) ; also sheet 6,9
HUB_!OVRCUR6: R32.1 S18.5(!FLG) ; also sheet 6,9
HUB_!OVRCUR7: R30.1 S16.5(!FLG) ; also sheet 6,9
HUB_!PWRON1: S8.1(I1) ; also sheet 6,9
HUB_!PWRON2: S7.1(I1) ; also sheet 6,9
HUB_!PWRON3: S9.1(I1) ; also sheet 6,9
HUB_!PWRON4: S11.1(I1) ; also sheet 6,9
HUB_!PWRON6: S12.1(I1) ; also sheet 6,9
HUB_!PWRON7: S10.1(I1) ; also sheet 6,9
MOD0_5V_METERED: C76.1 S13.2(IN) S13.3(IN) ; also sheet 1,4,9
MOD0_ISO_USB: S7.6(S) ; also sheet 3,7,9
MOD0_USB_!EN: S7.4(Z) S13.4(!EN)
MOD0_USB_VBUS: C77.1 C95.1 S13.6(OUT) S13.7(OUT) ; also sheet 2
MOD1_5V_METERED: C78.1 S14.2(IN) S14.3(IN) ; also sheet 1,4,9
MOD1_ISO_USB: S8.6(S) ; also sheet 3,7,9
MOD1_USB_!EN: S8.4(Z) S14.4(!EN)
MOD1_USB_VBUS: C79.1 C96.1 S14.6(OUT) S14.7(OUT) ; also sheet 2
MOD2_5V_METERED: C80.1 S15.2(IN) S15.3(IN) ; also sheet 1,4,9
MOD2_ISO_USB: S9.6(S) ; also sheet 3,7,9
MOD2_USB_!EN: S9.4(Z) S15.4(!EN)
MOD2_USB_VBUS: C81.1 C97.1 S15.6(OUT) S15.7(OUT) ; also sheet 2
MOD5_5V_METERED: C82.1 S16.2(IN) S16.3(IN) ; also sheet 1,4,9
MOD5_ISO_USB: S10.6(S) ; also sheet 3,7,9
MOD5_USB_!EN: S10.4(Z) S16.4(!EN)
MOD5_USB_VBUS: C83.1 C98.1 S16.6(OUT) S16.7(OUT) ; also sheet 2
MOD6_5V_METERED: C84.1 S17.2(IN) S17.3(IN) ; also sheet 1,4,9
MOD6_ISO_USB: S11.6(S) ; also sheet 3,7,9
MOD6_USB_!EN: S11.4(Z) S17.4(!EN)
MOD6_USB_VBUS: C85.1 C99.1 S17.6(OUT) S17.7(OUT) ; also sheet 2
MOD7_5V_METERED: C86.1 S18.2(IN) S18.3(IN) ; also sheet 1,4,9
MOD7_ISO_USB: S12.6(S) ; also sheet 3,7,9
MOD7_USB_!EN: S12.4(Z) S18.4(!EN)
MOD7_USB_VBUS: C87.1 C100.1 S18.6(OUT) S18.7(OUT) ; also sheet 2
VCC_BACKPLANE: C70.1 C71.1 C72.1 C73.1 C74.1 C75.1 R27.2 R28.2 R29.2 R30.2 R31.2 R32.2 S7.3(I0) S7.5(VCC) S8.3(I0) S8.5(VCC) S9.3(I0) S9.5(VCC) S10.3(I0) S10.5(VCC) S11.3(I0) S11.5(VCC) S12.3(I0) S12.5(VCC) ; also sheet 1,3,4,5,6,7,9

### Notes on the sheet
- USB
- Power switches & Iso Power Override

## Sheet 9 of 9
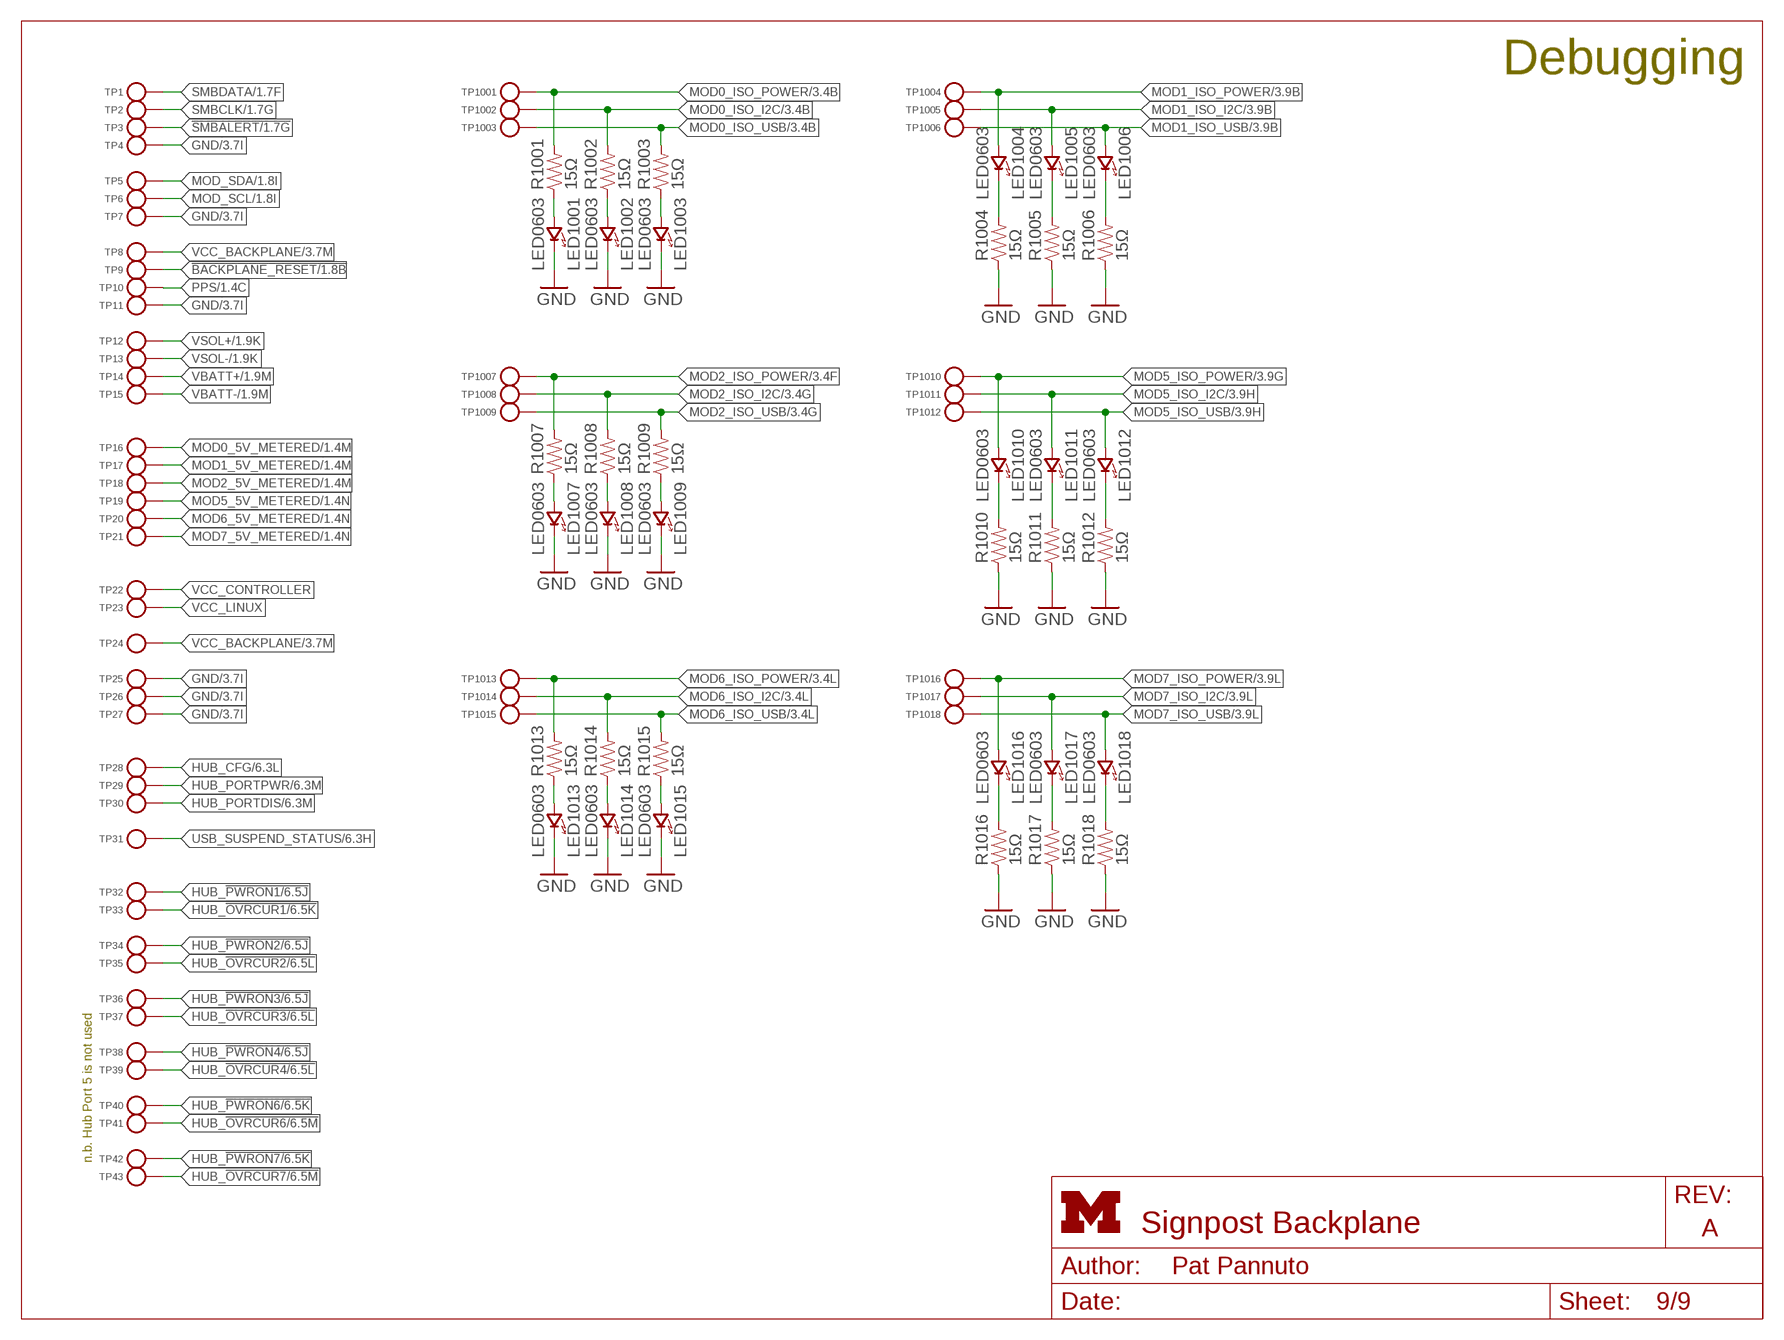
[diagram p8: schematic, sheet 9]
FRAME9 (LETTER_L_UMICH): HEIGHT: 8.5in; WIDTH: 11in

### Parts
LED1001  LED0603  [LED-0603]
LED1002  LED0603  [LED-0603]
LED1003  LED0603  [LED-0603]
LED1004  LED0603  [LED-0603]
LED1005  LED0603  [LED-0603]
LED1006  LED0603  [LED-0603]
LED1007  LED0603  [LED-0603]
LED1008  LED0603  [LED-0603]
LED1009  LED0603  [LED-0603]
LED1010  LED0603  [LED-0603]
LED1011  LED0603  [LED-0603]
LED1012  LED0603  [LED-0603]
LED1013  LED0603  [LED-0603]
LED1014  LED0603  [LED-0603]
LED1015  LED0603  [LED-0603]
LED1016  LED0603  [LED-0603]
LED1017  LED0603  [LED-0603]
LED1018  LED0603  [LED-0603]
R1001  15Ω  RESISTOR0603_RES  [0603-RES]
R1002  15Ω  RESISTOR0603_RES  [0603-RES]
R1003  15Ω  RESISTOR0603_RES  [0603-RES]
R1004  15Ω  RESISTOR0603_RES  [0603-RES]
R1005  15Ω  RESISTOR0603_RES  [0603-RES]
R1006  15Ω  RESISTOR0603_RES  [0603-RES]
R1007  15Ω  RESISTOR0603_RES  [0603-RES]
R1008  15Ω  RESISTOR0603_RES  [0603-RES]
R1009  15Ω  RESISTOR0603_RES  [0603-RES]
R1010  15Ω  RESISTOR0603_RES  [0603-RES]
R1011  15Ω  RESISTOR0603_RES  [0603-RES]
R1012  15Ω  RESISTOR0603_RES  [0603-RES]
R1013  15Ω  RESISTOR0603_RES  [0603-RES]
R1014  15Ω  RESISTOR0603_RES  [0603-RES]
R1015  15Ω  RESISTOR0603_RES  [0603-RES]
R1016  15Ω  RESISTOR0603_RES  [0603-RES]
R1017  15Ω  RESISTOR0603_RES  [0603-RES]
R1018  15Ω  RESISTOR0603_RES  [0603-RES]
TP1  TEST_POINT_0.040IN  [TESTPOINT_0.040IN]
TP2  TEST_POINT_0.040IN  [TESTPOINT_0.040IN]
TP3  TEST_POINT_0.040IN  [TESTPOINT_0.040IN]
TP4  TEST_POINT_0.040IN  [TESTPOINT_0.040IN]
TP5  TEST_POINT_0.040IN  [TESTPOINT_0.040IN]
TP6  TEST_POINT_0.040IN  [TESTPOINT_0.040IN]
TP7  TEST_POINT_0.040IN  [TESTPOINT_0.040IN]
TP8  TEST_POINT_0.040IN  [TESTPOINT_0.040IN]
TP9  TEST_POINT_0.040IN  [TESTPOINT_0.040IN]
TP10  TEST_POINT_0.040IN  [TESTPOINT_0.040IN]
TP11  TEST_POINT_0.040IN  [TESTPOINT_0.040IN]
TP12  TEST_POINT_0.040IN  [TESTPOINT_0.040IN]
TP13  TEST_POINT_0.040IN  [TESTPOINT_0.040IN]
TP14  TEST_POINT_0.040IN  [TESTPOINT_0.040IN]
TP15  TEST_POINT_0.040IN  [TESTPOINT_0.040IN]
TP16  TEST_POINT_0.040IN  [TESTPOINT_0.040IN]
TP17  TEST_POINT_0.040IN  [TESTPOINT_0.040IN]
TP18  TEST_POINT_0.040IN  [TESTPOINT_0.040IN]
TP19  TEST_POINT_0.040IN  [TESTPOINT_0.040IN]
TP20  TEST_POINT_0.040IN  [TESTPOINT_0.040IN]
TP21  TEST_POINT_0.040IN  [TESTPOINT_0.040IN]
TP22  TEST_POINT_0.040IN  [TESTPOINT_0.040IN]
TP23  TEST_POINT_0.040IN  [TESTPOINT_0.040IN]
TP24  TEST_POINT_0.040IN  [TESTPOINT_0.040IN]
TP25  TEST_POINT_0.040IN  [TESTPOINT_0.040IN]
TP26  TEST_POINT_0.040IN  [TESTPOINT_0.040IN]
TP27  TEST_POINT_0.040IN  [TESTPOINT_0.040IN]
TP28  TEST_POINT_0.040IN  [TESTPOINT_0.040IN]
TP29  TEST_POINT_0.040IN  [TESTPOINT_0.040IN]
TP30  TEST_POINT_0.040IN  [TESTPOINT_0.040IN]
TP31  TEST_POINT_0.040IN  [TESTPOINT_0.040IN]
TP32  TEST_POINT_0.040IN  [TESTPOINT_0.040IN]
TP33  TEST_POINT_0.040IN  [TESTPOINT_0.040IN]
TP34  TEST_POINT_0.040IN  [TESTPOINT_0.040IN]
TP35  TEST_POINT_0.040IN  [TESTPOINT_0.040IN]
TP36  TEST_POINT_0.040IN  [TESTPOINT_0.040IN]
TP37  TEST_POINT_0.040IN  [TESTPOINT_0.040IN]
TP38  TEST_POINT_0.040IN  [TESTPOINT_0.040IN]
TP39  TEST_POINT_0.040IN  [TESTPOINT_0.040IN]
TP40  TEST_POINT_0.040IN  [TESTPOINT_0.040IN]
TP41  TEST_POINT_0.040IN  [TESTPOINT_0.040IN]
TP42  TEST_POINT_0.040IN  [TESTPOINT_0.040IN]
TP43  TEST_POINT_0.040IN  [TESTPOINT_0.040IN]
TP1001  TEST_POINT_0.040IN  [TESTPOINT_0.040IN]
TP1002  TEST_POINT_0.040IN  [TESTPOINT_0.040IN]
TP1003  TEST_POINT_0.040IN  [TESTPOINT_0.040IN]
TP1004  TEST_POINT_0.040IN  [TESTPOINT_0.040IN]
TP1005  TEST_POINT_0.040IN  [TESTPOINT_0.040IN]
TP1006  TEST_POINT_0.040IN  [TESTPOINT_0.040IN]
TP1007  TEST_POINT_0.040IN  [TESTPOINT_0.040IN]
TP1008  TEST_POINT_0.040IN  [TESTPOINT_0.040IN]
TP1009  TEST_POINT_0.040IN  [TESTPOINT_0.040IN]
TP1010  TEST_POINT_0.040IN  [TESTPOINT_0.040IN]
TP1011  TEST_POINT_0.040IN  [TESTPOINT_0.040IN]
TP1012  TEST_POINT_0.040IN  [TESTPOINT_0.040IN]
TP1013  TEST_POINT_0.040IN  [TESTPOINT_0.040IN]
TP1014  TEST_POINT_0.040IN  [TESTPOINT_0.040IN]
TP1015  TEST_POINT_0.040IN  [TESTPOINT_0.040IN]
TP1016  TEST_POINT_0.040IN  [TESTPOINT_0.040IN]
TP1017  TEST_POINT_0.040IN  [TESTPOINT_0.040IN]
TP1018  TEST_POINT_0.040IN  [TESTPOINT_0.040IN]

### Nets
!BACKPLANE_RESET: TP9.TESTPOINT ; also sheet 1,3,6
!SMBALERT: TP3.TESTPOINT ; also sheet 1
GND: LED1001.C(CATHODE) LED1002.C(CATHODE) LED1003.C(CATHODE) LED1007.C(CATHODE) LED1008.C(CATHODE) LED1009.C(CATHODE) LED1013.C(CATHODE) LED1014.C(CATHODE) LED1015.C(CATHODE) R1004.1 R1005.1 R1006.1 R1010.1 R1011.1 R1012.1 R1016.1 R1017.1 R1018.1 TP4.TESTPOINT TP7.TESTPOINT TP11.TESTPOINT TP25.TESTPOINT TP26.TESTPOINT TP27.TESTPOINT ; also sheet 1,2,3,4,5,6,7,8
HUB_!OVRCUR1: TP33.TESTPOINT ; also sheet 6,8
HUB_!OVRCUR2: TP35.TESTPOINT ; also sheet 6,8
HUB_!OVRCUR3: TP37.TESTPOINT ; also sheet 6,8
HUB_!OVRCUR4: TP39.TESTPOINT ; also sheet 6,8
HUB_!OVRCUR6: TP41.TESTPOINT ; also sheet 6,8
HUB_!OVRCUR7: TP43.TESTPOINT ; also sheet 6,8
HUB_!PWRON1: TP32.TESTPOINT ; also sheet 6,8
HUB_!PWRON2: TP34.TESTPOINT ; also sheet 6,8
HUB_!PWRON3: TP36.TESTPOINT ; also sheet 6,8
HUB_!PWRON4: TP38.TESTPOINT ; also sheet 6,8
HUB_!PWRON6: TP40.TESTPOINT ; also sheet 6,8
HUB_!PWRON7: TP42.TESTPOINT ; also sheet 6,8
HUB_CFG: TP28.TESTPOINT ; also sheet 6
HUB_PORTDIS: TP30.TESTPOINT ; also sheet 6
HUB_PORTPWR: TP29.TESTPOINT ; also sheet 6
MOD0_5V_METERED: TP16.TESTPOINT ; also sheet 1,4,8
MOD0_ISO_I2C: R1002.2 TP1002.TESTPOINT ; also sheet 3,4
MOD0_ISO_POWER: R1001.2 TP1001.TESTPOINT ; also sheet 3,4
MOD0_ISO_USB: R1003.2 TP1003.TESTPOINT ; also sheet 3,7,8
MOD1_5V_METERED: TP17.TESTPOINT ; also sheet 1,4,8
MOD1_ISO_I2C: LED1005.A(ANODE) TP1005.TESTPOINT ; also sheet 3,4
MOD1_ISO_POWER: LED1004.A(ANODE) TP1004.TESTPOINT ; also sheet 3,4
MOD1_ISO_USB: LED1006.A(ANODE) TP1006.TESTPOINT ; also sheet 3,7,8
MOD2_5V_METERED: TP18.TESTPOINT ; also sheet 1,4,8
MOD2_ISO_I2C: R1008.2 TP1008.TESTPOINT ; also sheet 3,4
MOD2_ISO_POWER: R1007.2 TP1007.TESTPOINT ; also sheet 3,4
MOD2_ISO_USB: R1009.2 TP1009.TESTPOINT ; also sheet 3,7,8
MOD5_5V_METERED: TP19.TESTPOINT ; also sheet 1,4,8
MOD5_ISO_I2C: LED1011.A(ANODE) TP1011.TESTPOINT ; also sheet 3,4
MOD5_ISO_POWER: LED1010.A(ANODE) TP1010.TESTPOINT ; also sheet 3,4
MOD5_ISO_USB: LED1012.A(ANODE) TP1012.TESTPOINT ; also sheet 3,7,8
MOD6_5V_METERED: TP20.TESTPOINT ; also sheet 1,4,8
MOD6_ISO_I2C: R1014.2 TP1014.TESTPOINT ; also sheet 3,4
MOD6_ISO_POWER: R1013.2 TP1013.TESTPOINT ; also sheet 3,4
MOD6_ISO_USB: R1015.2 TP1015.TESTPOINT ; also sheet 3,7,8
MOD7_5V_METERED: TP21.TESTPOINT ; also sheet 1,4,8
MOD7_ISO_I2C: LED1017.A(ANODE) TP1017.TESTPOINT ; also sheet 3,4
MOD7_ISO_POWER: LED1016.A(ANODE) TP1016.TESTPOINT ; also sheet 3,4
MOD7_ISO_USB: LED1018.A(ANODE) TP1018.TESTPOINT ; also sheet 3,7,8
MOD_SCL: TP6.TESTPOINT ; also sheet 1,4
MOD_SDA: TP5.TESTPOINT ; also sheet 1,4
N$1: LED1001.A(ANODE) R1001.1
N$2: LED1002.A(ANODE) R1002.1
N$3: LED1003.A(ANODE) R1003.1
N$4: LED1007.A(ANODE) R1007.1
N$5: LED1008.A(ANODE) R1008.1
N$6: LED1009.A(ANODE) R1009.1
N$7: LED1013.A(ANODE) R1013.1
N$8: LED1014.A(ANODE) R1014.1
N$9: LED1015.A(ANODE) R1015.1
N$10: LED1004.C(CATHODE) R1004.2
N$11: LED1005.C(CATHODE) R1005.2
N$13: LED1006.C(CATHODE) R1006.2
N$15: LED1010.C(CATHODE) R1010.2
N$16: LED1011.C(CATHODE) R1011.2
N$28: LED1012.C(CATHODE) R1012.2
N$29: LED1016.C(CATHODE) R1016.2
N$30: LED1017.C(CATHODE) R1017.2
N$32: LED1018.C(CATHODE) R1018.2
PPS: TP10.TESTPOINT ; also sheet 1,5
SMBCLK: TP2.TESTPOINT ; also sheet 1,3
SMBDATA: TP1.TESTPOINT ; also sheet 1,3
USB_SUSPEND_STATUS: TP31.TESTPOINT ; also sheet 6
VBATT+: TP14.TESTPOINT ; also sheet 1
VBATT-: TP15.TESTPOINT ; also sheet 1
VCC_BACKPLANE: TP8.TESTPOINT TP24.TESTPOINT ; also sheet 1,3,4,5,6,7,8
VCC_CONTROLLER: TP22.TESTPOINT ; also sheet 1
VCC_LINUX: TP23.TESTPOINT ; also sheet 1
VSOL+: TP12.TESTPOINT ; also sheet 1
VSOL-: TP13.TESTPOINT ; also sheet 1

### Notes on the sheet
- Debugging
- n.b. Hub Port 5 is not used

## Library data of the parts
C1 C2 = passives:CAPACITOR: 0402 Capacitor; DIGIKEY: 1276-1023-1-ND
C3-C94 = passives:CAPACITOR: 0402 Capacitor
C95-C100 = passives:CAPACITOR: 0402 Capacitor; DIGIKEY: 1276-3367-1-ND
D1-D4 = signpost:SN75240-TSSOP: TVS Diodes [suggested for TI USB Hub] (2 array); DIGIKEY: 296-6596-1-ND
J0 J1 J2 J5-J7 = signpost:BACKPLANE_GENERIC_MODULE: Signpost generic module recepticle; DIGIKEY: S9195-ND
J3 = signpost:BACKPLANE_CONTROLLER_MODULE: Signpost controller recepticle; DIGIKEY: S9197-ND , S9194-ND
J4 = signpost:BACKPLANE_POWER_MODULE: Signpost power module recepticle; DIGIKEY: S9197-ND
J8 J9 = connector:SCREW_TERMINAL: PCB terminal block 5mm; DIGIKEY: 277-1667-ND
LED1001-LED1018 = leds:LED: LED
LOGO1 = logos:UMICH_SOLID
R1-R80 R1001-R1018 = passives:RESISTOR: Resistor
S1-S6 = signpost:SIP3240X: High power (2.4 A) high-side switch; DIGIKEY: SIP32402ADNP-T1GE4CT-ND
S7-S12 = signpost:NC7SZ157: MUX; DIGIKEY: NC7SZ157P6XCT-ND
S13-S18 = signpost:AP2401MP: USB Power Switch; DIGIKEY: AP2401MP-13DICT-ND
TP1-TP43 TP1001-TP1018 = headers:TEST_POINT_0.040IN: 0.040in Test Point; DIGIKEY: 5001K-ND
U1 = signpost:TUSB2077A: Full Speed USB Hub - 7 Port; DIGIKEY: 296-37871-1-ND
U2-U7 = signpost:FXMA2102: Dual Supply, 2-Bit Voltage Translator / Buffer / Repeater / Isolator for I2C; DIGIKEY: FXMA2102UMXCT-ND
U8-U19 = signpost:SN74LVC2T45: Bidirectional Buffer / Level Converter 2 Circuits; DIGIKEY: 296-17014-1-ND
U20-U25 = signpost:TS3USB30E: USB Mux with OE control and ESD; DIGIKEY: 296-24684-1-ND
U26-U31 = signpost:MCP23008: GPIO Extender via I2C - 8 Pin; DIGIKEY: MCP23008T-E/SOCT-ND
Y1 = crystals:ABMM: Low-Profile SMD crystal; DIGIKEY: 535-10156-1-ND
